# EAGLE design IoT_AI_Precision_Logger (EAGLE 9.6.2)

## Sheet 1 of 4: ADC, Buff Amp, VREF Circuits
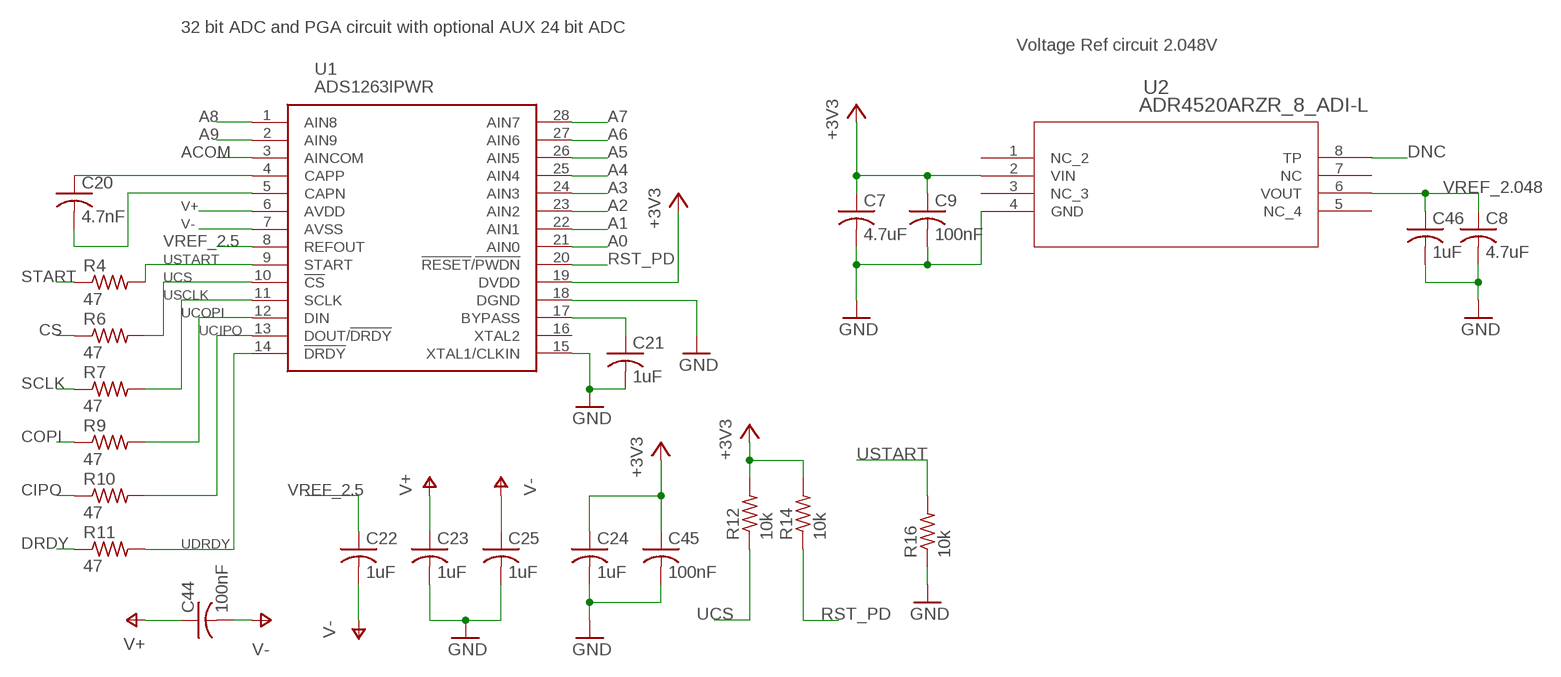
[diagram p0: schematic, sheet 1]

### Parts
C7  4.7uF  C-USC0603  [C0603]
C8  4.7uF  C-USC0603  [C0603]
C9  100nF  C-USC0603  [C0603]
C20  4.7nF  C-USC0603  [C0603]
C21  1uF  C-USC0603  [C0603]
C22  1uF  C-USC0603  [C0603]
C23  1uF  C-USC0603  [C0603]
C24  1uF  C-USC0603  [C0603]
C25  1uF  C-USC0603  [C0603]
C44  100nF  C-USC0603  [C0603]
C45  100nF  C-USC0603  [C0603]
C46  1uF  C-USC0603  [C0603]
R4  47  R-US_R0603  [R0603]
R6  47  R-US_R0603  [R0603]
R7  47  R-US_R0603  [R0603]
R9  47  R-US_R0603  [R0603]
R10  47  R-US_R0603  [R0603]
R11  47  R-US_R0603  [R0603]
R12  10k  R-US_R0603  [R0603]
R14  10k  R-US_R0603  [R0603]
R16  10k  R-US_R0603  [R0603]
U1  ADS1263IPWR  [SOP65P640X120-28N]
U2  ADR4520ARZR_8_ADI-L  [R_8_ADI-L]

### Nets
+3V3: C7.1 C9.1 C24.1 C45.1 R12.2 R14.2 U1.19(DVDD) U2.2(VIN) ; also sheet 2,3,4
A0: U1.21(AIN0) ; also sheet 3
A1: U1.22(AIN1) ; also sheet 3
A2: U1.23(AIN2) ; also sheet 3
A3: U1.24(AIN3) ; also sheet 3
A4: U1.25(AIN4) ; also sheet 3
A5: U1.26(AIN5) ; also sheet 3
A6: U1.27(AIN6) ; also sheet 3
A7: U1.28(AIN7) ; also sheet 3
A8: U1.1(AIN8) ; also sheet 3
A9: U1.2(AIN9) ; also sheet 3
ACOM: U1.3(AINCOM) ; also sheet 3
CIPO: R10.1 ; also sheet 3,4
COPI: R9.1 ; also sheet 4
CS: R6.1 ; also sheet 4
DNC: U2.8(TP)
DRDY: R11.1 ; also sheet 4
GND: C7.2 C8.2 C9.2 C21.2 C23.2 C24.2 C25.2 C45.2 C46.2 R16.1 U1.15(XTAL1/CLKIN) U1.18(DGND) U2.4(GND) ; also sheet 2,3,4
N$8: C20.1 U1.4(CAPP)
N$9: C20.2 U1.5(CAPN)
N$28: C21.1 U1.17(BYPASS)
RST_PD: R14.1 U1.20(!RESET!/!PWDN) ; also sheet 4
SCLK: R7.1 ; also sheet 4
START: R4.1 ; also sheet 4
UCIPO: R10.2 U1.13(DOUT/!DRDY)
UCOPI: R9.2 U1.12(DIN) ; also sheet 3
UCS: R6.2 R12.1 U1.10(!CS)
UDRDY: R11.2 U1.14(!DRDY)
USCLK: R7.2 U1.11(SCLK) ; also sheet 3
USTART: R4.2 R16.2 U1.9(START)
V+: C23.1 C44.1 U1.6(AVDD) ; also sheet 2
V-: C22.2 C25.1 C44.2 U1.7(AVSS) ; also sheet 2,3
VREF_2.5: C22.1 U1.8(REFOUT) ; also sheet 3
VREF_2.048: C8.1 C46.1 U2.6(VOUT) ; also sheet 3
Unconnected: U1.16(XTAL2) U2.1(NC_2) U2.3(NC_3) U2.5(NC_4) U2.7(NC)

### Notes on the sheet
- 32 bit ADC and PGA circuit with optional AUX 24 bit ADC
- Voltage Ref circuit 2.048V

## Sheet 2 of 4: Onboard Power Circuits
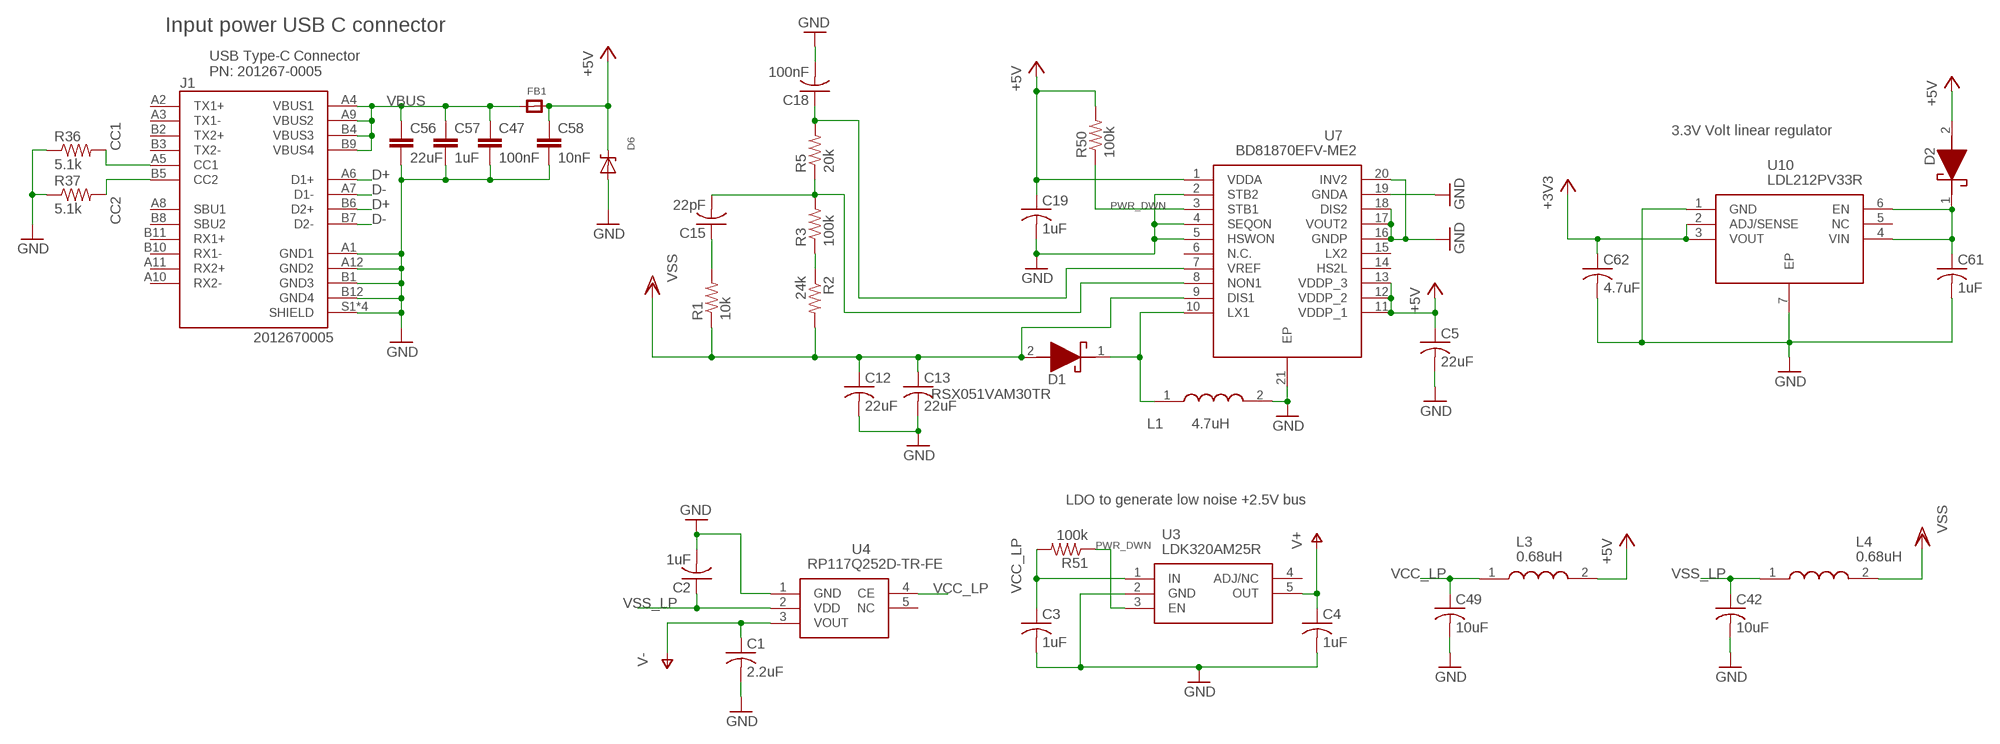
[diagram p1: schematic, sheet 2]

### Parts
C1  2.2uF  C-USC0603  [C0603]
C2  1uF  C-USC0603  [C0603]
C3  1uF  C-USC0603  [C0603]
C4  1uF  C-USC0603  [C0603]
C5  22uF  C-USC0603  [C0603]
C12  22uF  C-USC0603  [C0603]
C13  22uF  C-USC0603  [C0603]
C15  22pF  C-USC0603  [C0603]
C18  100nF  C-USC0603  [C0603]
C19  1uF  C-USC0603  [C0603]
C42  10uF  C-USC0603  [C0603]
C47  100nF  C-EUC0603  [C0603]
C49  10uF  C-USC0603  [C0603]
C56  22uF  C-EUC0603  [C0603]
C57  1uF  C-EUC0603  [C0603]
C58  10nF  C-EUC0603  [C0603]
C61  1uF  C-USC0603  [C0603]
C62  4.7uF  C-USC0603  [C0603]
D1  RSX051VAM30TR  [RSX051VAM30TR]
D2  CUS10S30,H3F  [CUZ10V]
D6  DDZ5V6ASF  [DDZ5V6ASF]
FB1  FERRITE_0603  [_0603]
J1  2012670005  [MOLEX_2012670005]
L1  4.7uH  LQM21PN4R7MGSD  [LQM21PHR47NG0D]
L3  0.68uH  MLF2012DR68MT000  [INDC2012X145N]
L4  0.68uH  MLF2012DR68MT000  [INDC2012X145N]
R1  10k  R-US_R0603  [R0603]
R2  24k  R-US_R0603  [R0603]
R3  100k  R-US_R0603  [R0603]
R5  20k  R-US_R0603  [R0603]
R36  5.1k  R-US_R0603  [R0603]
R37  5.1k  R-US_R0603  [R0603]
R50  100k  R-US_R0603  [R0603]
R51  100k  R-US_R0603  [R0603]
U3  LDK320AM25R  [SOT95P280X125-5N]
U4  RP117Q252D-TR-FE  [SOT65P210X110-5N]
U7  BD81870EFV-ME2  [SOP65P640X100-21N]
U10  LDL212PV33R  [SON50P200X200X80-7N]

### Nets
+3V3: C62.1 U10.2(ADJ/SENSE) U10.3(VOUT) ; also sheet 1,3,4
+5V: C5.1 C19.1 C58.1 D2.2(A) D6.P$2(C) FB1.2 L3.2 R50.2 U7.1(VDDA) U7.11(VDDP_1) U7.12(VDDP_2) U7.13(VDDP_3) ; also sheet 4
CC1: J1.A5(CC1) R36.2
CC2: J1.B5(CC2) R37.2
D+: J1.A6(D1+) J1.B6(D2+) ; also sheet 4
D-: J1.A7(D1-) J1.B7(D2-) ; also sheet 4
GND: C1.2 C2.2 C3.2 C4.2 C5.2 C12.2 C13.2 C18.2 C19.2 C42.2 C47.2 C49.2 C56.2 C57.2 C58.2 C61.2 C62.2 D6.P$1(A) J1.A1(GND1) J1.A12(GND2) J1.B1(GND3) J1.B12(GND4) J1.S1(SHIELD) J1.S2(SHIELD) J1.S3(SHIELD) J1.S4(SHIELD) L1.2 R36.1 R37.1 U3.2(GND) U4.1(GND) U7.2(STB2) U7.4(SEQON) U7.5(HSWON) U7.16(GNDP) U7.17(VOUT2) U7.18(DIS2) U7.19(GNDA) U7.20(INV2) U7.21(EP) U10.1(GND) U10.7(EP) ; also sheet 1,3,4
N$1: C61.1 D2.1(K) U10.4(VIN) U10.6(EN)
N$4: C15.2 R3.2 R5.1 U7.8(NON1)
N$5: D1.1(K) L1.1 U7.10(LX1)
N$6: C18.1 R5.2 U7.7(VREF)
N$7: C15.1 R1.2
N$11: R2.1 R3.1
PWR_DWN: R50.1 R51.1 U3.3(EN) U7.3(STB1) ; also sheet 4
V+: C4.1 U3.5(OUT) ; also sheet 1
V-: C1.1 U4.3(VOUT) ; also sheet 1,3
VBUS: C47.1 C56.1 C57.1 FB1.1 J1.A4(VBUS1) J1.A9(VBUS2) J1.B4(VBUS3) J1.B9(VBUS4) ; also sheet 3
VCC_LP: C3.1 C49.1 L3.1 R51.2 U3.1(IN) U4.4(CE)
VSS: C12.1 C13.1 D1.2(A) L4.2 R1.1 R2.2 U7.9(DIS1)
VSS_LP: C2.1 C42.1 L4.1 U4.2(VDD)
Unconnected: J1.A2(TX1+) J1.A3(TX1-) J1.A8(SBU1) J1.A10(RX2-) J1.A11(RX2+) J1.B2(TX2+) J1.B3(TX2-) J1.B8(SBU2) J1.B10(RX1-) J1.B11(RX1+) U3.4(ADJ/NC) U4.5(NC) U7.6(N.C.) U7.14(HS2L) U7.15(LX2) U10.5(NC)

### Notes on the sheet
- Input power USB C connector
- USB Type-C Connector
  PN: 201267-0005
- 3.3V Volt linear regulator
- LDO to generate low noise +2.5V bus

## Sheet 3 of 4: Connectors and Switching
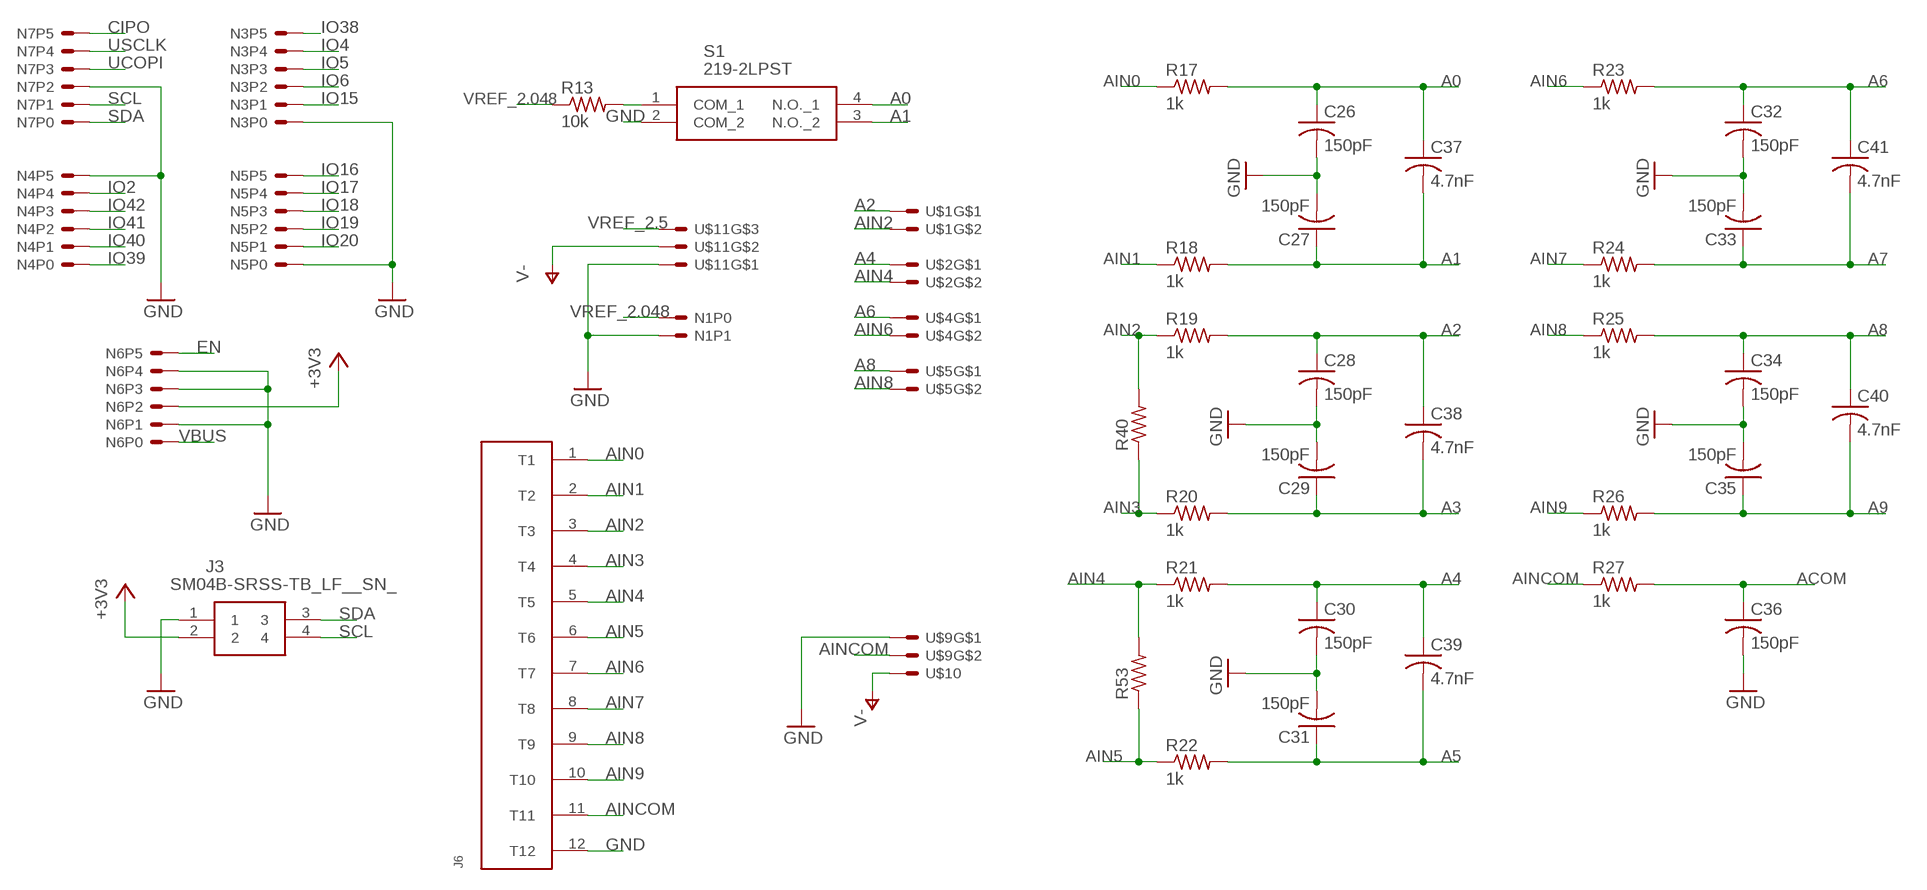
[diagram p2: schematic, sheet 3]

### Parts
C26  150pF  C-USC0603  [C0603]
C27  150pF  C-USC0603  [C0603]
C28  150pF  C-USC0603  [C0603]
C29  150pF  C-USC0603  [C0603]
C30  150pF  C-USC0603  [C0603]
C31  150pF  C-USC0603  [C0603]
C32  150pF  C-USC0603  [C0603]
C33  150pF  C-USC0603  [C0603]
C34  150pF  C-USC0603  [C0603]
C35  150pF  C-USC0603  [C0603]
C36  150pF  C-USC0603  [C0603]
C37  4.7nF  C-USC0603  [C0603]
C38  4.7nF  C-USC0603  [C0603]
C39  4.7nF  C-USC0603  [C0603]
C40  4.7nF  C-USC0603  [C0603]
C41  4.7nF  C-USC0603  [C0603]
J3  SM04B-SRSS-TB_LF__SN_  [SM04B-SRSS-TB(LFSN)]
J6  BARRIER_BLOCK_12POS  [BARRIER_BLOCK_12POS]
N1  2PINHEADER  [2PINHEADER]
N3  6PINHEADER  [6PINHEADER]
N4  6PINHEADER  [6PINHEADER]
N5  6PINHEADER  [6PINHEADER]
N6  6PINHEADER  [6PINHEADER]
N7  6PINHEADER  [6PINHEADER]
R13  10k  R-US_R0603  [R0603]
R17  1k  R-US_R0603  [R0603]
R18  1k  R-US_R0603  [R0603]
R19  1k  R-US_R0603  [R0603]
R20  1k  R-US_R0603  [R0603]
R21  1k  R-US_R0603  [R0603]
R22  1k  R-US_R0603  [R0603]
R23  1k  R-US_R0603  [R0603]
R24  1k  R-US_R0603  [R0603]
R25  1k  R-US_R0603  [R0603]
R26  1k  R-US_R0603  [R0603]
R27  1k  R-US_R0603  [R0603]
R40  R-US_R1206  [R1206]
R53  R-US_R1206  [R1206]
S1  219-2LPST  [2192LPST]
U$1  2PINHEADER_S  [2PINHEADER_S]
U$2  2PINHEADER_S  [2PINHEADER_S]
U$4  2PINHEADER_S  [2PINHEADER_S]
U$5  2PINHEADER_S  [2PINHEADER_S]
U$9  2PINHEADER_S  [2PINHEADER_S]
U$10  1PINHEADER_S  [1PINHEADER_S]
U$11  3PINHEADER  [3PINHEADER]

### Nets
+3V3: J3.2 N6.P2 ; also sheet 1,2,4
A0: C26.1 C37.1 R17.2 S1.4(N.O._1) ; also sheet 1
A1: C27.1 C37.2 R18.2 S1.3(N.O._2) ; also sheet 1
A2: C28.1 C38.1 R19.2 U$1.N0 ; also sheet 1
A3: C29.1 C38.2 R20.2 ; also sheet 1
A4: C30.1 C39.1 R21.2 U$2.N0 ; also sheet 1
A5: C31.1 C39.2 R22.2 ; also sheet 1
A6: C32.1 C41.1 R23.2 U$4.N0 ; also sheet 1
A7: C33.1 C41.2 R24.2 ; also sheet 1
A8: C34.1 C40.1 R25.2 U$5.N0 ; also sheet 1
A9: C35.1 C40.2 R26.2 ; also sheet 1
ACOM: C36.1 R27.2 ; also sheet 1
AIN0: J6.1(T1) R17.1
AIN1: J6.2(T2) R18.1
AIN2: J6.3(T3) R19.1 R40.2 U$1.N1
AIN3: J6.4(T4) R20.1 R40.1
AIN4: J6.5(T5) R21.1 R53.2 U$2.N1
AIN5: J6.6(T6) R22.1 R53.1
AIN6: J6.7(T7) R23.1 U$4.N1
AIN7: J6.8(T8) R24.1
AIN8: J6.9(T9) R25.1 U$5.N1
AIN9: J6.10(T10) R26.1
AINCOM: J6.11(T11) R27.1 U$9.N1
CIPO: N7.P5 ; also sheet 1,4
EN: N6.P5 ; also sheet 4
GND: C26.2 C27.2 C28.2 C29.2 C30.2 C31.2 C32.2 C33.2 C34.2 C35.2 C36.2 J3.1 J6.12(T12) N1.P1 N3.P0 N4.P5 N5.P0 N6.P1 N6.P3 N6.P4 N7.P2 S1.2(COM_2) U$9.N0 U$11.N0 ; also sheet 1,2,4
IO2: N4.P4 ; also sheet 4
IO4: N3.P4 ; also sheet 4
IO5: N3.P3 ; also sheet 4
IO6: N3.P2 ; also sheet 4
IO15: N3.P1 ; also sheet 4
IO16: N5.P5 ; also sheet 4
IO17: N5.P4 ; also sheet 4
IO18: N5.P3 ; also sheet 4
IO19: N5.P2 ; also sheet 4
IO20: N5.P1 ; also sheet 4
IO38: N3.P5 ; also sheet 4
IO39: N4.P0 ; also sheet 4
IO40: N4.P1 ; also sheet 4
IO41: N4.P2 ; also sheet 4
IO42: N4.P3 ; also sheet 4
N$2: R13.2 S1.1(COM_1)
SCL: J3.4 N7.P1 ; also sheet 4
SDA: J3.3 N7.P0 ; also sheet 4
UCOPI: N7.P3 ; also sheet 1
USCLK: N7.P4 ; also sheet 1
V-: U$10.P$1(S) U$11.N1 ; also sheet 1,2
VBUS: N6.P0 ; also sheet 2
VREF_2.5: U$11.N2 ; also sheet 1
VREF_2.048: N1.P0 R13.1 ; also sheet 1

## Sheet 4 of 4: ESP32 Circuit
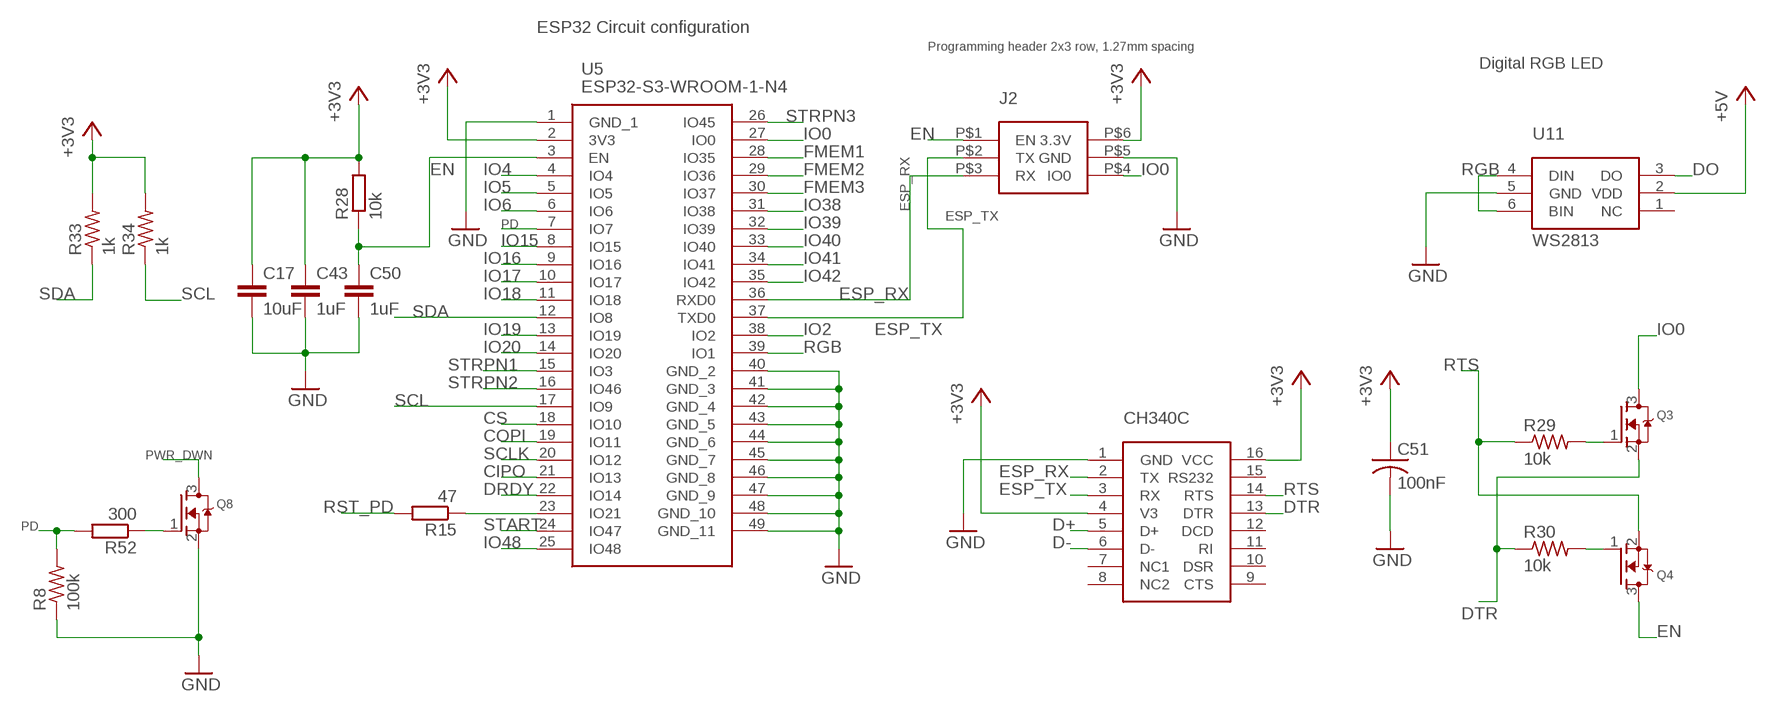
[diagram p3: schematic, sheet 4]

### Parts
C17  10uF  C-EUC0603  [C0603]
C43  1uF  C-EUC0603  [C0603]
C50  1uF  C-EUC0603  [C0603]
C51  100nF  C-USC0603  [C0603]
J2  ESP-PROG_HEADER  [2X3_1.27_HEADER]
Q3  MOSFET-NREFLOW  [SOT23-R]
Q4  MOSFET-NREFLOW  [SOT23-R]
Q8  MOSFET-NREFLOW  [SOT23-R]
R8  100k  R-US_R0603  [R0603]
R15  47  R-EU_R0603  [R0603]
R28  10k  R-EU_R0603  [R0603]
R29  10k  R-US_R0603  [R0603]
R30  10k  R-US_R0603  [R0603]
R33  1k  R-US_R0603  [R0603]
R34  1k  R-US_R0603  [R0603]
R52  300  R-EU_R0603  [R0603]
U5  ESP32-S3-WROOM-1-N4  [ESP32S3WROOM1N4]
U6  CH340C  [SOIC16]
U11  WS2813  [WS2813]

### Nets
+3V3: C17.1 C43.1 C51.1 J2.P$6(3.3V) R28.2 R33.2 R34.2 U5.2(3V3) U6.4(V3) U6.16(VCC) ; also sheet 1,2,3
+5V: U11.2(VDD) ; also sheet 2
CIPO: U5.21(IO13) ; also sheet 1,3
COPI: U5.19(IO11) ; also sheet 1
CS: U5.18(IO10) ; also sheet 1
D+: U6.5(D+) ; also sheet 2
D-: U6.6(D-) ; also sheet 2
DO: U11.3(DO)
DRDY: U5.22(IO14) ; also sheet 1
DTR: Q3.2(S) R30.1 U6.13(DTR)
EN: C50.1 J2.P$1(EN) Q4.3(D) R28.1 U5.3(EN) ; also sheet 3
ESP_RX: J2.P$3(RX) U5.36(RXD0) U6.2(TX)
ESP_TX: J2.P$2(TX) U5.37(TXD0) U6.3(RX)
FMEM1: U5.28(IO35)
FMEM2: U5.29(IO36)
FMEM3: U5.30(IO37)
GND: C17.2 C43.2 C50.2 C51.2 J2.P$5(GND) Q8.2(S) R8.1 U5.1(GND_1) U5.40(GND_2) U5.41(GND_3) U5.42(GND_4) U5.43(GND_5) U5.44(GND_6) U5.45(GND_7) U5.46(GND_8) U5.47(GND_9) U5.48(GND_10) U5.49(GND_11) U6.1(GND) U11.5(GND) ; also sheet 1,2,3
IO0: J2.P$4(IO0) Q3.3(D) U5.27(IO0)
IO2: U5.38(IO2) ; also sheet 3
IO4: U5.4(IO4) ; also sheet 3
IO5: U5.5(IO5) ; also sheet 3
IO6: U5.6(IO6) ; also sheet 3
IO15: U5.8(IO15) ; also sheet 3
IO16: U5.9(IO16) ; also sheet 3
IO17: U5.10(IO17) ; also sheet 3
IO18: U5.11(IO18) ; also sheet 3
IO19: U5.13(IO19) ; also sheet 3
IO20: U5.14(IO20) ; also sheet 3
IO38: U5.31(IO38) ; also sheet 3
IO39: U5.32(IO39) ; also sheet 3
IO40: U5.33(IO40) ; also sheet 3
IO41: U5.34(IO41) ; also sheet 3
IO42: U5.35(IO42) ; also sheet 3
IO48: U5.25(IO48)
N$3: Q4.1(G) R30.2
N$10: Q3.1(G) R29.2
N$17: R15.1 U5.23(IO21)
N$24: Q8.1(G) R52.1
PD: R8.2 R52.2 U5.7(IO7)
PWR_DWN: Q8.3(D) ; also sheet 2
RGB: U5.39(IO1) U11.4(DIN) U11.6(BIN)
RST_PD: R15.2 ; also sheet 1
RTS: Q4.2(S) R29.1 U6.14(RTS)
SCL: R34.1 U5.17(IO9) ; also sheet 3
SCLK: U5.20(IO12) ; also sheet 1
SDA: R33.1 U5.12(IO8) ; also sheet 3
START: U5.24(IO47) ; also sheet 1
STRPN1: U5.15(IO3)
STRPN2: U5.16(IO46)
STRPN3: U5.26(IO45)
Unconnected: U6.7(NC1) U6.8(NC2) U6.9(CTS) U6.10(DSR) U6.11(RI) U6.12(DCD) U6.15(RS232) U11.1(NC)

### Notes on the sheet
- ESP32 Circuit configuration
- Programming header 2x3 row, 1.27mm spacing
- Digital RGB LED
- CH340C

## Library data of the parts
C1-C5 C7-C9 C12 C13 C15 C18-C42 C44-C46 C49 C51 C61 C62 = rcl:C-US: CAPACITOR, American symbol; SPICEPREFIX: C
C17 C43 C47 C50 C56-C58 = rcl:C-EU: CAPACITOR, European symbol; SPICEPREFIX: C
D1 = SamacSys_Parts:RSX051VAM30TR: ROHM 30V 500mA, SiC Schottky Diode, 2-Pin SOD-323HE RSX051VAM30TR; DESCRIPTION: ROHM 30V 500mA, SiC Schottky Diode, 2-Pin SOD-323HE RSX051VAM30TR; HEIGHT: 0.8mm; MANUFACTURER_NAME: ROHM Semiconductor; MANUFACTURER_PART_NUMBER: RSX051VAM30TR; MOUSER_PART_NUMBER: 755-RSX051VAM30TR; MOUSER_PRICE-STOCK: https://www.mouser.co.uk/ProductDetail/ROHM-Semiconductor/RSX051VAM30TR?qs=4v%252BiZTmLVHH6gyykIHF0SA%3D%3D
D2 = SamacSys_Parts:CUS10S30,H3F: Schottky Diodes & Rectifiers Single High-speed switching; DESCRIPTION: Schottky Diodes & Rectifiers Single High-speed switching; HEIGHT: 1.1mm; MANUFACTURER_NAME: Toshiba; MANUFACTURER_PART_NUMBER: CUS10S30,H3F; MOUSER_PART_NUMBER: 757-CUS10S30H3F; MOUSER_PRICE-STOCK: https://www.mouser.co.uk/ProductDetail/Toshiba/CUS10S30H3F?qs=cW4DzVrAanO4Xm6ySrHr7g%3D%3D
D6 = ForceTronics:DDZ5V6ASF: DDZ5V6ASF 5.42 Zener Diode
FB1 = microbuilder:FERRITE: Ferrite Bead
J1 = 2012670005:2012670005: USB-C (USB TYPE-C) USB 3.1 (USB 3.1 Gen 2, Superspeed+) Receptacle Connector 24 Position Surface Mount, Right Angle; Through Hole Check availability; AVAILABILITY: In Stock; DESCRIPTION: USB-C (USB TYPE-C) USB 3.2 Gen 2 (USB 3.1 Gen 2, Superspeed + (USB 3.1)) Receptacle Connector 24 Position Surface Mount, Right Angle; Through Hole; MF: Molex; MP: 2012670005; PACKAGE: None; PRICE: None; PURCHASE-URL: https://pricing.snapeda.com/search/part/2012670005/?ref=eda
J2 = ForceTronics:ESP-PROG_HEADER: 2x3 programming header for the ESP32 with 1.27mm spacing
J3 = SamacSys_Parts:SM04B-SRSS-TB_LF__SN_: JST (JAPAN SOLDERLESS TERMINALS) - SM04B-SRSS-TB(LF)(SN) - CONNECTOR, HEADER, SMT, R/A, 1MM, 4WAY Source: Datasheet; DESCRIPTION: JST (JAPAN SOLDERLESS TERMINALS) - SM04B-SRSS-TB(LF)(SN) - CONNECTOR, HEADER, SMT, R/A, 1MM, 4WAY; HEIGHT: mm; MANUFACTURER_NAME: JST (JAPAN SOLDERLESS TERMINALS); MANUFACTURER_PART_NUMBER: SM04B-SRSS-TB(LF)(SN); MOUSER_PART_NUMBER: 306-SM04BSRSSTBLFSN; MOUSER_PRICE-STOCK: https://www.mouser.co.uk/ProductDetail/JST-Commercial/SM04B-SRSS-TBLFSN?qs=cdbOS8ANM9B3FdyA6cNU2A%3D%3D
J6 = ForceTronics-ForceTronics:BARRIER_BLOCK_12POS: 1 Row 12 positon 7.62mm pin spacing Barrier Bar from Amazon
L1 = SamacSys_Parts:LQM21PN4R7MGSD: LQM21PN_GS Series Inductor 4.7uH +/-20% 0805 (2012); DESCRIPTION: LQM21PN_GS Series Inductor 4.7uH +/-20% 0805 (2012); HEIGHT: 1mm; MANUFACTURER_NAME: Murata Electronics; MANUFACTURER_PART_NUMBER: LQM21PN4R7MGSD; MOUSER_PART_NUMBER: 81-LQM21PN4R7MGSD; MOUSER_PRICE-STOCK: https://www.mouser.co.uk/ProductDetail/Murata-Electronics/LQM21PN4R7MGSD?qs=Gufeu08L%2Fl2uzbzo%2FrY4bg%3D%3D
L3 L4 = SamacSys_Parts:MLF2012DR68MT000: SMD / SMT Inductors (Coils), L=0.68?H, L x W x T :; DESCRIPTION: SMD / SMT Inductors (Coils), L=0.68?H, L x W x T :; HEIGHT: 1.45mm; MANUFACTURER_NAME: TDK; MANUFACTURER_PART_NUMBER: MLF2012DR68MT000
N1 = ForceTronics:2PINHEADER
N3-N7 = ForceTronics:6PINHEADER
Q3 Q4 Q8 = microbuilder:MOSFET-N: N-Channel Mosfet LEGEND VDS: Voltage Drain-Source ID: Drain Current RDS(ON): Drain-Source On-State Resistance VGS(TH): Gate-Source Threshold Voltage CISS: Drain-Source Input Capacitance SOT-23 Name VDS ID RDS(ON) VGS(TH) CISS Order Number 2N7002E 60V 260mA 2.5 Ohm 2.5V @ 250uA 26.7pF @ 25V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
R1-R14 R16-R27 R29 R30 R33 R34 R36 R37 R40 R50 R51 R53 = rcl:R-US_: RESISTOR, American symbol; SPICEPREFIX: R
R15 R28 R52 = rcl:R-EU_: RESISTOR, European symbol; SPICEPREFIX: R
S1 = SamacSys_Parts:219-2LPST: Dip Switch SPST 2 Position Surface Mount Slide (Standard) Actuator 100mA 20VDC Source: Datasheet; DESCRIPTION: Dip Switch SPST 2 Position Surface Mount Slide (Standard) Actuator 100mA 20VDC; HEIGHT: mm; MANUFACTURER_NAME: CTS; MANUFACTURER_PART_NUMBER: 219-2LPST; MOUSER_PART_NUMBER: 774-2192LPST; MOUSER_PRICE-STOCK: https://www.mouser.co.uk/ProductDetail/CTS-Electronic-Components/219-2LPST?qs=qNzHFtQhdJ96rtXqLWSQzw%3D%3D
U1 = SamacSys_Parts:ADS1263IPWR: 32-Bit, 38kSPS, 10-Ch Delta-Sigma ADC w/ PGA, Voltage Reference, and Aux ADC for Factory Automation Source: Datasheet; DESCRIPTION: 32-Bit, 38kSPS, 10-Ch Delta-Sigma ADC w/ PGA, Voltage Reference, and Aux ADC for Factory Automation; HEIGHT: 1.2mm; MANUFACTURER_NAME: Texas Instruments; MANUFACTURER_PART_NUMBER: ADS1263IPWR; MOUSER_PART_NUMBER: 595-ADS1263IPWR; MOUSER_PRICE-STOCK: https://www.mouser.co.uk/ProductDetail/Texas-Instruments/ADS1263IPWR?qs=GURawfaeGuAEKG2KPkczsw%3D%3D
U2 = ForceTronics:ADR4520ARZ; COPYRIGHT: Copyright (C) 2025 Ultra Librarian. All rights reserved.; MANUFACTURER_PART_NUMBER: ADR4520ARZ; MFR_NAME: Analog Devices Inc
U3 = SamacSys_Parts:LDK320AM25R: 200 mA low quiescent current and high PSRR voltage regulator Source: Datasheet; DESCRIPTION: 200 mA low quiescent current and high PSRR voltage regulator; HEIGHT: 1.25mm; MANUFACTURER_NAME: STMicroelectronics; MANUFACTURER_PART_NUMBER: LDK320AM25R; MOUSER_PART_NUMBER: 511-LDK320AM25R; MOUSER_PRICE-STOCK: https://www.mouser.co.uk/ProductDetail/STMicroelectronics/LDK320AM25R?qs=wd5RIQLrsJiQNxEkfV2I5w%3D%3D
U4 = SamacSys_Parts:RP117Q252D-TR-FE: LDO Voltage Regulators 100 mA LDO Regulator Source: Datasheet; DESCRIPTION: LDO Voltage Regulators 100 mA LDO Regulator; HEIGHT: 1.1mm; MANUFACTURER_NAME: Nisshinbo; MANUFACTURER_PART_NUMBER: RP117Q252D-TR-FE; MOUSER_PART_NUMBER: 848-RP117Q252D-TR-FE; MOUSER_PRICE-STOCK: https://www.mouser.co.uk/ProductDetail/Nisshinbo/RP117Q252D-TR-FE?qs=0lQeLiL1qyb%252B39Gkjsmryg%3D%3D
U5 = ESP32-S3-WROOM-1-N4:ESP32-S3-WROOM-1-N4: WiFi Modules - 802.11 [Engineering Samples] SMD Module, ESP32-S3, 4 MB SPI Flash, PCB Antenna Source: Datasheet; DESCRIPTION: WiFi Modules - 802.11 [Engineering Samples] SMD Module, ESP32-S3, 4 MB SPI Flash, PCB Antenna; HEIGHT: 3.25mm; MANUFACTURER_NAME: Espressif Systems; MANUFACTURER_PART_NUMBER: ESP32-S3-WROOM-1-N4; MOUSER_PART_NUMBER: 356-ESP32-S3WROOM1N4; MOUSER_PRICE-STOCK: https://www.mouser.co.uk/ProductDetail/Espressif-Systems/ESP32-S3-WROOM-1-N4?qs=Li%252BoUPsLEnsO%2FkiJOUK0FQ%3D%3D
U6 = ForceTronics:CH340C: CH340C IC that converts USB to UART
U7 = SamacSys_Parts:BD81870EFV-ME2: ROHM - BD81870EFV-ME2 - DC/DC Switching Regulator, Inverting, Step Up, 2 Output, 2.5V to 5.5VIn, 18V out, 2.1MHz, HTSSOP-20 Source: Datasheet; DESCRIPTION: ROHM - BD81870EFV-ME2 - DC/DC Switching Regulator, Inverting, Step Up, 2 Output, 2.5V to 5.5VIn, 18V out, 2.1MHz, HTSSOP-20; HEIGHT: 1mm; MANUFACTURER_NAME: ROHM Semiconductor; MANUFACTURER_PART_NUMBER: BD81870EFV-ME2; MOUSER_PART_NUMBER: 755-BD81870EFV-ME2; MOUSER_PRICE-STOCK: https://www.mouser.co.uk/ProductDetail/ROHM-Semiconductor/BD81870EFV-ME2/?qs=HXFqYaX1Q2wm5IkeUd4YKg%3D%3D
U10 = SamacSys_Parts:LDL212PV33R: LDO Voltage Regulators VFDFPN 6 2x2x0.75 PITCH 0.5 Source: Datasheet; DESCRIPTION: LDO Voltage Regulators VFDFPN 6 2x2x0.75 PITCH 0.5; HEIGHT: 0.8mm; MANUFACTURER_NAME: STMicroelectronics; MANUFACTURER_PART_NUMBER: LDL212PV33R; MOUSER_PART_NUMBER: 511-LDL212PV33R; MOUSER_PRICE-STOCK: https://www.mouser.co.uk/ProductDetail/STMicroelectronics/LDL212PV33R?qs=5aG0NVq1C4xm%252BbuBme%252BLZw%3D%3D
U11 = ForceTronics:WS2813: WS2813 Intelligent control integrated LED light source Device
U$1 U$2 U$4 U$5 U$9 = ForceTronics:2PINHEADER_S: 2 pin header with round copper
U$10 = ForceTronics:1PINHEADER_S: 1 pin header with round pad
U$11 = ForceTronics:3PINHEADER: 3 pin header with oval copper

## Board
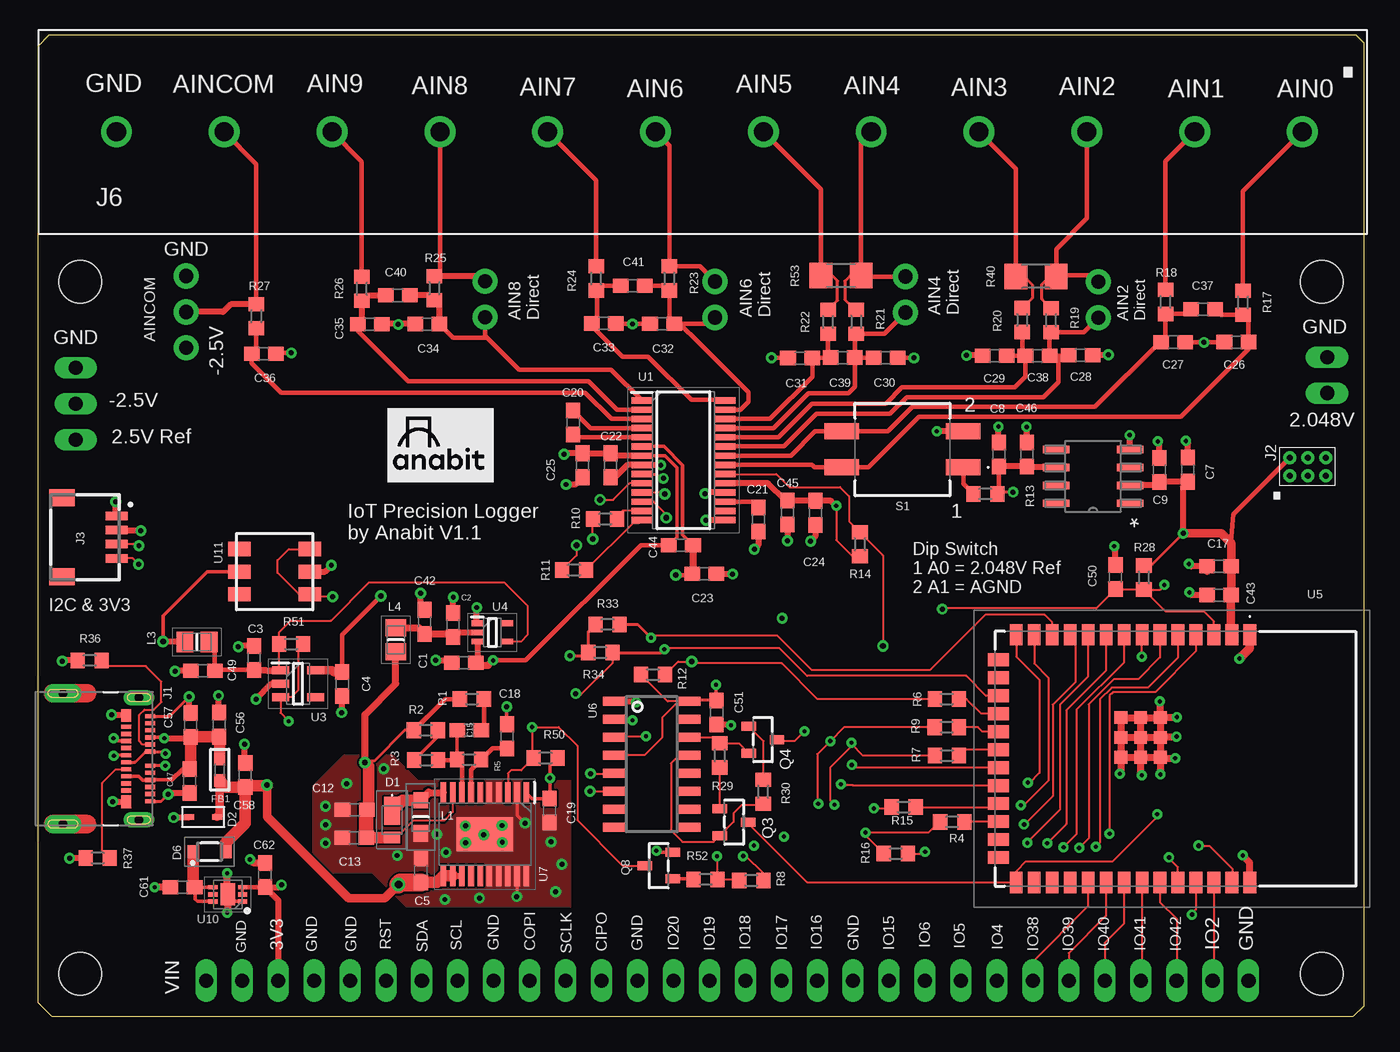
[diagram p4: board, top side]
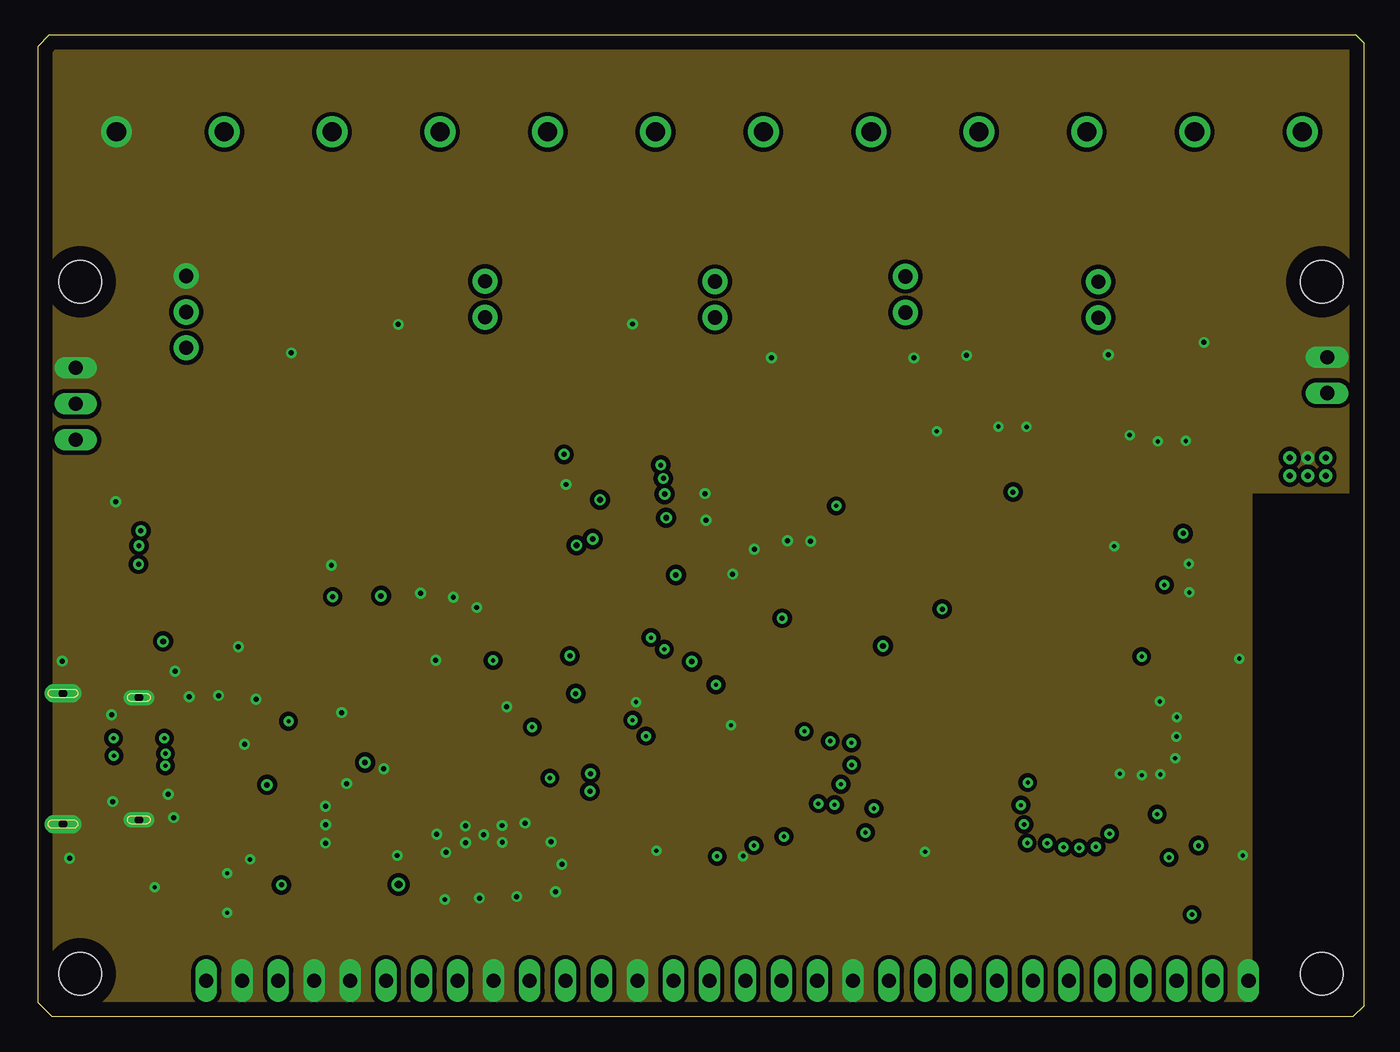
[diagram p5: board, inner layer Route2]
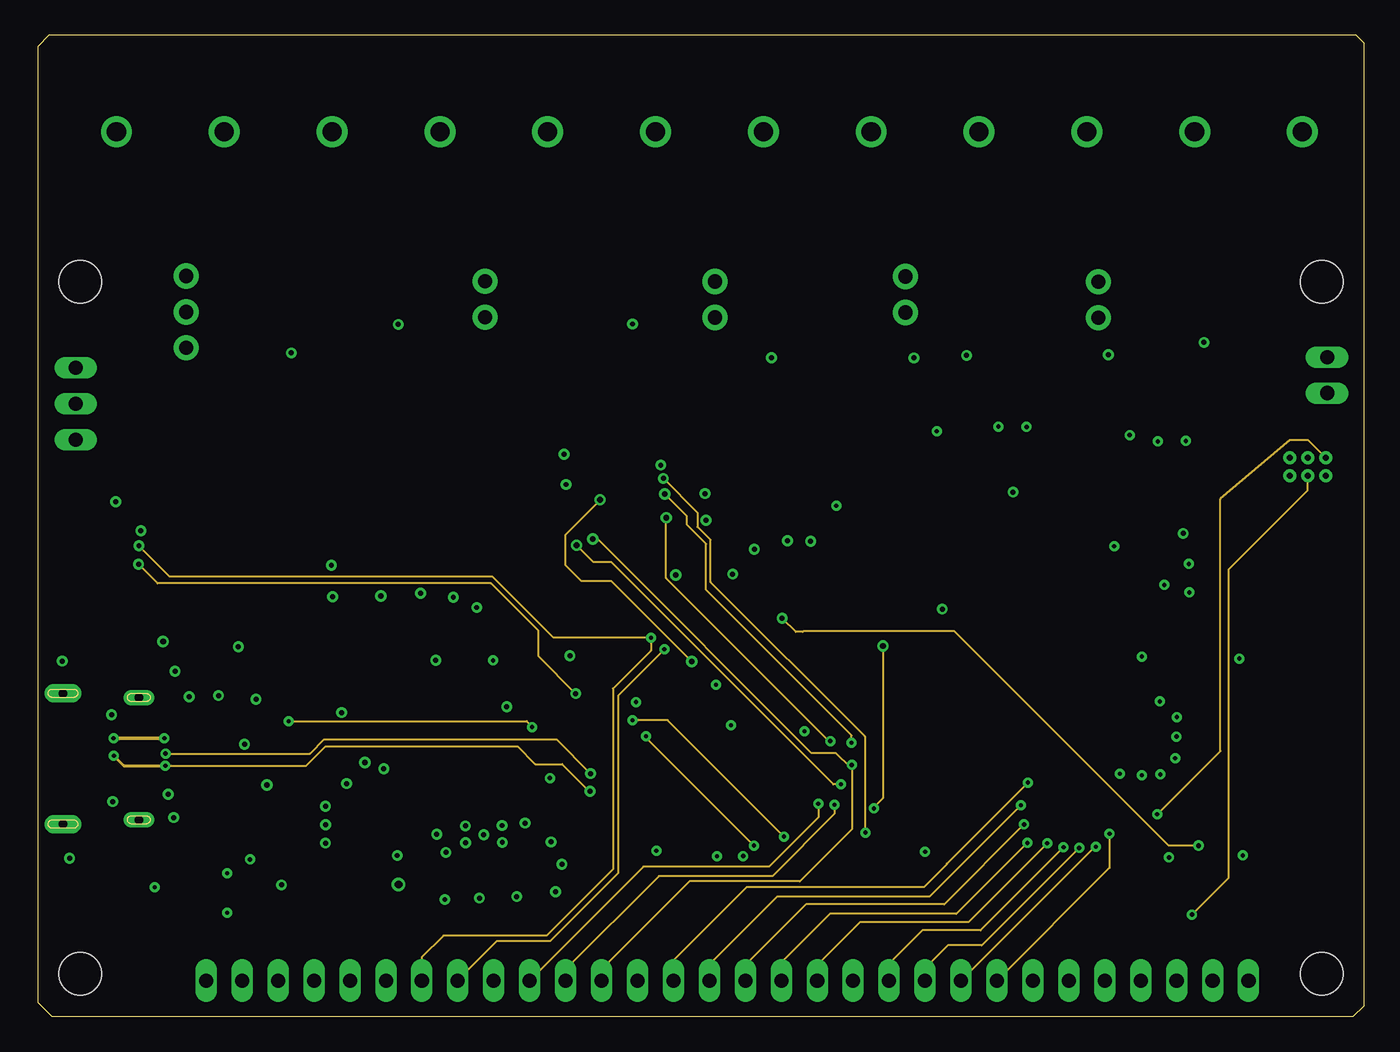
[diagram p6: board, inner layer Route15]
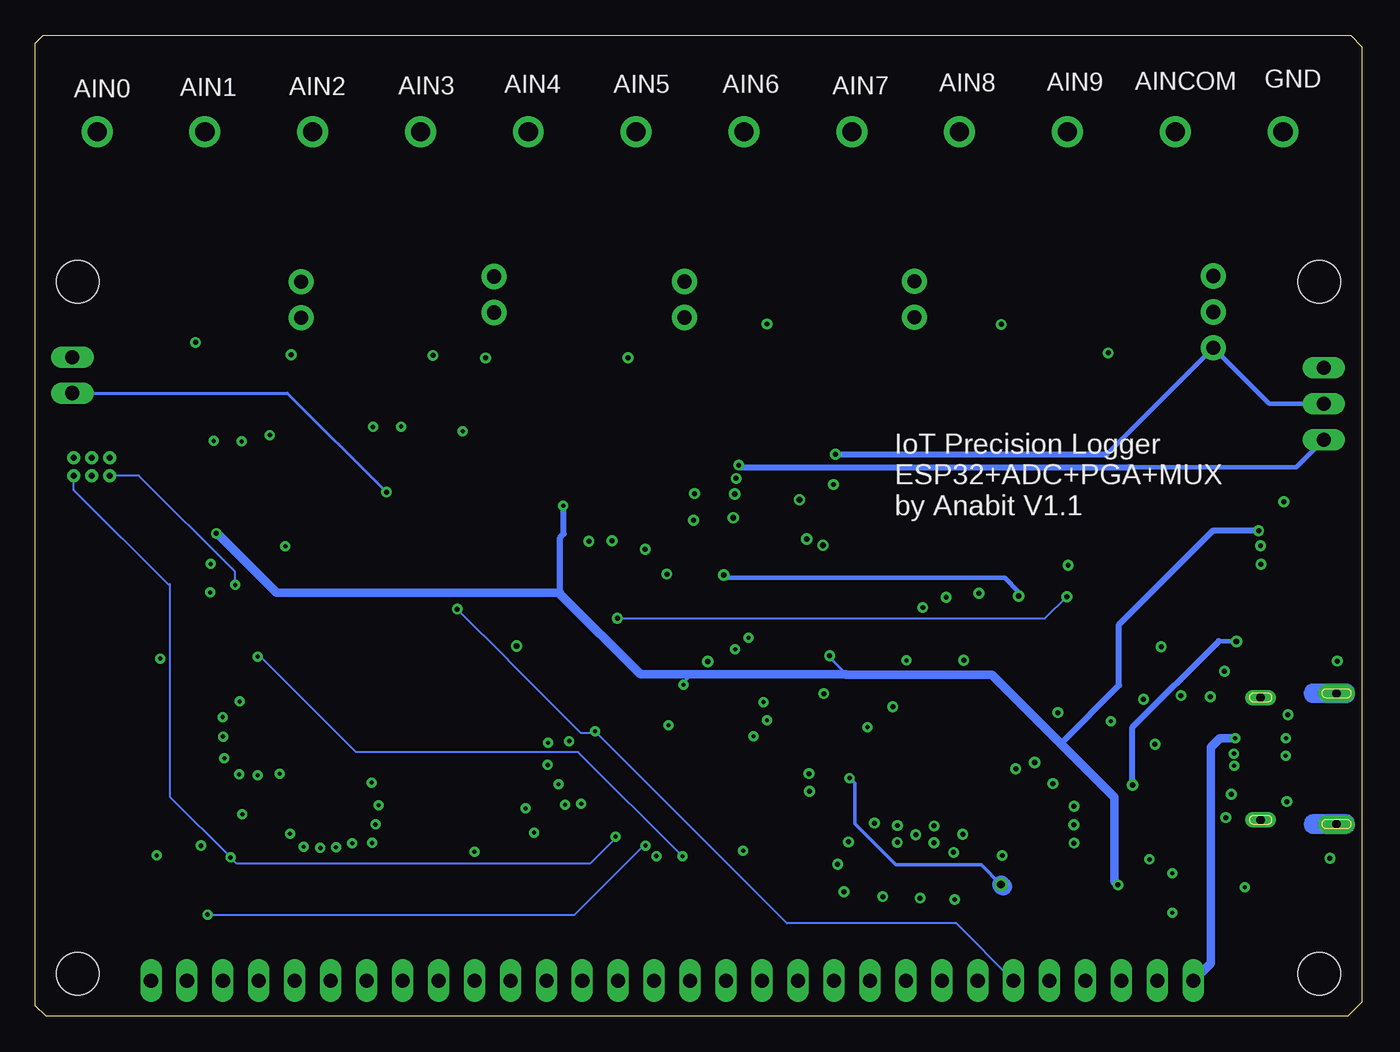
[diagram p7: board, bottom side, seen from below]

Size 93.74 x 69.3 mm. Coordinates in mm from the lower left corner, seen from the top.
Outline: 93.19,69.3 0.79,69.3 0,68.51 0,0.99 0.99,0 92.99,0 93.74,0.75 93.74,68.75 93.19,69.3
Copper layers (1+2*15+16): Top 0.035mm / dielectric 0.5mm / Route2 0.035mm / dielectric 0.75mm / Route15 0.035mm / dielectric 0.75mm / Bottom 0.035mm
Design rules "default *": minimum track width 6mil, minimum drill 0.3mm, track to track 6mil, track to pad 6mil, pad to pad 6mil, via to via 6mil, smd to smd 6mil, copper to edge 40mil, drill to drill 6mil, minimum pad ring 10mil, minimum via ring 8mil, stop-mask expansion 4mil, vias tented up to drill 0mil, thermal gap 10mil
Holes 3 mm at 2.99,51.9 90.75,51.9 2.99,3 90.75,3

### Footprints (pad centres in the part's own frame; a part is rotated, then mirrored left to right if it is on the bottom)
C0603 = smd 1.1 x 1: 1 -0.85,0; 2 0.85,0
RSX051VAM30TR = smd 1.1 x 2: 1 0,0.65 | smd 1.1 x 0.8: 2 0,-1.25
CUZ10V = smd 0.9 x 0.8: 1 0,-1.15; 2 0,1.15
DDZ5V6ASF = smd 0.71 x 0.41: P$1 0,0; P$2 1.99,0
_0603 = smd 0.9 x 0.8: 1 -0.762,0; 2 0.762,0
MOLEX_2012670005 = smd 0.3 x 0.7: A1 -3,0.81; A2 -2.5,0.81; A3 -2,0.81; A4 -1.5,0.81; A5 -1,0.81; A6 -0.5,0.81; A7 0.5,0.81; A8 1,0.81; A9 1.5,0.81; A10 2,0.81; A11 2.5,0.81; A12 3,0.81; B2 2.25,-0.89; B3 1.75,-0.89; B4 1.25,-0.89; B5 0.75,-0.89; B6 0.25,-0.89; B7 -0.25,-0.89; B8 -0.75,-0.89; B9 -1.25,-0.89; B10 -1.75,-0.89; B11 -2.25,-0.89 | smd 0.9 x 0.7: B1 3.05,-0.89; B12 -3.05,-0.89 | drill 0.6 pad 1.1 long: S1 -4.32,0; S2 4.32,0 | drill 0.6 pad 1.3 long: S3 -4.62,-5.36; S4 4.62,-5.36
2X3_1.27_HEADER = drill 0.419 pad 0.75: P$1 0,0; P$2 1.27,0; P$3 2.54,0; P$4 2.54,1.27; P$5 1.27,1.27; P$6 0,1.27
SM04B-SRSS-TB(LFSN) = smd 0.6 x 1.55: 1 1.5,4.661; 2 2.5,4.661; 3 3.5,4.661; 4 4.5,4.661 | smd 1.2 x 1.8: 5 0.2,0.786; 6 5.8,0.786
BARRIER_BLOCK_12POS = drill 1.35 pad 2.184: 1 0,0; 2 7.62,0; 3 15.24,0; 4 22.86,0; 5 30.48,0; 6 38.1,0; 7 45.72,0; 8 53.34,0; 9 60.96,0; 10 68.58,0; 11 76.2,0; 12 83.82,0
LQM21PHR47NG0D = smd 1.15 x 1: 1 -1.175,0; 2 1.175,0
INDC2012X145N = smd 1.2 x 1.45: 1 -0.85,0; 2 0.85,0
2PINHEADER = drill 1 long: P0 -1.27,0; P1 1.27,0
6PINHEADER = drill 1 long: P0 1.27,-1.778; P1 3.81,-1.778; P2 6.35,-1.778; P3 8.89,-1.778; P4 11.43,-1.778; P5 13.97,-1.778
SOT23-R = smd 0.635 x 1.016: 1 -0.95,-1; 2 0.95,-1; 3 0,1
R0603 = smd 1 x 1.1: 1 -0.85,0; 2 0.85,0
R1206 = smd 1.6 x 1.803: 1 -1.422,0; 2 1.422,0
2192LPST = smd 1.13 x 2.44: 1 -1.27,-4.3; 2 1.27,-4.3; 3 1.27,4.3; 4 -1.27,4.3
SOP65P640X120-28N = smd 1.475 x 0.45: 1 -2.938,4.225; 2 -2.938,3.575; 3 -2.938,2.925; 4 -2.938,2.275; 5 -2.938,1.625; 6 -2.938,0.975; 7 -2.938,0.325; 8 -2.938,-0.325; 9 -2.938,-0.975; 10 -2.938,-1.625; 11 -2.938,-2.275; 12 -2.938,-2.925; 13 -2.938,-3.575; 14 -2.938,-4.225; 15 2.938,-4.225; 16 2.938,-3.575; 17 2.938,-2.925; 18 2.938,-2.275; 19 2.938,-1.625; 20 2.938,-0.975; 21 2.938,-0.325; 22 2.938,0.325; 23 2.938,0.975; 24 2.938,1.625; 25 2.938,2.275; 26 2.938,2.925; 27 2.938,3.575; 28 2.938,4.225
R_8_ADI-L = smd 1.876 x 0.508: 1 -2.613,1.905; 2 -2.613,0.635; 3 -2.613,-0.635; 4 -2.613,-1.905; 5 2.613,-1.905; 6 2.613,-0.635; 7 2.613,0.635; 8 2.613,1.905
SOT95P280X125-5N = smd 1.2 x 0.55: 1 -1.25,0.95; 2 -1.25,0; 3 -1.25,-0.95; 4 1.25,-0.95; 5 1.25,0.95
SOT65P210X110-5N = smd 0.85 x 0.4: 1 -1.05,0.65; 2 -1.05,0; 3 -1.05,-0.65; 4 1.05,-0.65; 5 1.05,0.65
ESP32S3WROOM1N4 = smd 1.5 x 0.9: 1 -8.75,5.26; 2 -8.75,3.99; 3 -8.75,2.72; 4 -8.75,1.45; 5 -8.75,0.18; 6 -8.75,-1.09; 7 -8.75,-2.36; 8 -8.75,-3.63; 9 -8.75,-4.9; 10 -8.75,-6.17; 11 -8.75,-7.44; 12 -8.75,-8.71; 13 -8.75,-9.98; 14 -8.75,-11.25; 27 8.75,-11.25; 28 8.75,-9.98; 29 8.75,-8.71; 30 8.75,-7.44; 31 8.75,-6.17; 32 8.75,-4.9; 33 8.75,-3.63; 34 8.75,-2.36; 35 8.75,-1.09; 36 8.75,0.18; 37 8.75,1.45; 38 8.75,2.72; 39 8.75,3.99; 40 8.75,5.26 | smd 0.9 x 1.5: 15 -6.985,-12.5; 16 -5.715,-12.5; 17 -4.445,-12.5; 18 -3.175,-12.5; 19 -1.905,-12.5; 20 -0.635,-12.5; 21 0.635,-12.5; 22 1.905,-12.5; 23 3.175,-12.5; 24 4.445,-12.5; 25 5.715,-12.5; 26 6.985,-12.5 | smd 0.9 x 0.9: 41 -1.5,-2.46; 42 -0.1,-2.46; 43 -0.1,-1.06; 44 -1.5,-1.06; 45 -2.9,-1.06; 46 -2.9,-2.46; 47 -2.9,-3.86; 48 -1.5,-3.86; 49 -0.1,-3.86
SOIC16 = smd 0.635 x 1.524: 1 -4.445,-2.695; 2 -3.175,-2.695; 3 -1.905,-2.695; 4 -0.635,-2.695; 5 0.635,-2.695; 6 1.905,-2.695; 7 3.175,-2.695; 8 4.445,-2.695; 9 4.445,2.695; 10 3.175,2.695; 11 1.905,2.695; 12 0.635,2.695; 13 -0.635,2.695; 14 -1.905,2.695; 15 -3.175,2.695; 16 -4.445,2.695
SOP65P640X100-21N = smd 1.475 x 0.4: 1 -2.938,2.925; 2 -2.938,2.275; 3 -2.938,1.625; 4 -2.938,0.975; 5 -2.938,0.325; 6 -2.938,-0.325; 7 -2.938,-0.975; 8 -2.938,-1.625; 9 -2.938,-2.275; 10 -2.938,-2.925; 11 2.938,-2.925; 12 2.938,-2.275; 13 2.938,-1.625; 14 2.938,-0.975; 15 2.938,-0.325; 16 2.938,0.325; 17 2.938,0.975; 18 2.938,1.625; 19 2.938,2.275; 20 2.938,2.925 | smd 2.4 x 4: 21 0,0
SON50P200X200X80-7N = smd 0.65 x 0.3: 1 -1.05,0.5; 2 -1.05,0; 3 -1.05,-0.5; 4 1.05,-0.5; 5 1.05,0; 6 1.05,0.5 | smd 1.02 x 1.55: 7 0,0
WS2813 = smd 1.6 x 1: 1 5.2,1.1; 2 5.2,2.7; 3 5.2,4.3; 4 0.2,4.3; 5 0.2,2.7; 6 0.2,1.1
2PINHEADER_S = drill 1 pad 1.778: N0 2.59,0.056; N1 0.05,0.056
1PINHEADER_S = drill 1 pad 1.778: P$1 1.27,1.27
3PINHEADER = drill 1 long: N0 1.27,1.27; N1 3.81,1.27; N2 6.35,1.27

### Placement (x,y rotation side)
C1  30.12,24.98 180 top
C2  29.35,27.65 90 top
C3  15.29,25.32 90 top
C4  21.52,23.47 270 top
C5  27.08,10.31 90 top
C7  81.28,38.62 90 top
C8  67.92,39.7 90 top
C9  79.27,38.6 90 top
C12  22.39,14.59 180 top
C13  22.37,12.62 180 top
C15  30.49,20.22 180 top
C17  83.49,31.79 180 top
C18  33.16,19.78 90 top
C19  36.17,14.53 270 top
C20  37.84,41.94 270 top
C21  50.93,35.11 270 top
C22  40.49,38.93 90 top
C23  47.11,31.26 0 top
C24  54.96,35.57 270 top
C25  38.5,38.93 270 top
C26  84.71,47.64 180 top
C27  80.25,47.63 0 top
C28  73.69,46.7 0 top
C29  67.62,46.66 180 top
C30  59.92,46.53 0 top
C31  53.87,46.51 180 top
C32  44.12,48.93 180 top
C33  40,48.94 0 top
C34  27.52,48.91 180 top
C35  23.46,48.89 0 top
C36  15.97,46.8 0 top
C37  82.36,49.96 180 top
C38  70.65,46.66 180 top
C39  56.89,46.54 180 top
C40  25.45,50.93 180 top
C41  42.04,51.61 180 top
C42  27.35,27.87 90 top
C43  83.48,29.76 180 top
C44  45.46,33.29 180 top
C45  52.98,35.59 270 top
C46  69.91,39.7 90 top
C47  10.74,16.62 270 top
C49  11.66,24.41 180 top
C50  76.17,31.03 90 top
C51  47.98,21.47 270 top
C56  12.82,20.6 90 top
C57  10.81,20.57 90 top
C58  14.67,17.04 90 top
C61  10.24,9.11 180 top
C62  16.06,9.97 90 top
D1  25.04,13.87 0 top
D2  12.14,11.63 270 top
D6  10.69,14.08 0 top
FB1  12.86,17.42 270 top
J1  7.14,18.2 270 top
J2  88.48,38.19 0 top
J3  0.91,36.85 270 top
J6  89.38,62.48 180 top
L1  27.07,14.08 270 top
L3  11.25,26.44 180 top
L4  25.3,26.6 270 top
N1  91.13,45.3 90 top
N3  56.35,4.3 0 top
N4  71.6,4.3 0 top
N5  41.12,4.3 0 top
N6  10.64,4.3 0 top
N7  25.87,4.3 0 top
Q3  49.21,13.72 270 top
Q4  51.24,19.54 270 top
Q8  43.89,10.65 90 top
R1  30.68,22.41 0 top
R2  27.43,20.21 180 top
R3  27.44,18.1 0 top
R4  64.63,13.73 180 top
R5  30.49,18.13 0 top
R6  64.25,22.41 180 top
R7  64.25,18.42 180 top
R8  50.43,9.59 180 top
R9  64.24,20.42 180 top
R10  40.1,35.13 0 top
R11  37.9,31.53 0 top
R12  43.48,24.14 180 top
R13  66.97,36.91 180 top
R14  58.11,33.34 270 top
R15  61.2,14.78 180 top
R16  60.64,11.49 180 top
R17  85.18,50.42 270 top
R18  79.7,50.47 270 top
R19  71.61,49.17 270 top
R20  69.58,49.19 270 top
R21  57.85,49.07 270 top
R22  55.85,49.06 270 top
R23  44.64,52.13 270 top
R24  39.46,52.13 270 top
R25  28.04,51.44 270 top
R26  22.9,51.4 270 top
R27  15.45,49.45 270 top
R28  78.17,31 90 top
R29  48.2,18.43 270 top
R30  51.26,15.87 90 top
R33  40.26,27.69 180 top
R34  39.76,25.7 180 top
R36  3.67,25.14 0 top
R37  4.24,11.18 0 top
R40  70.55,52.27 0 top
R50  35.88,18.25 0 top
R51  17.91,26.29 180 top
R52  47.2,9.67 0 top
R53  56.77,52.33 0 top
S1  61.11,40.05 90 top
U1  45.63,39.28 0 top
U2  74.58,38.14 180 top
U3  18.4,23.49 0 top
U4  32.12,27.12 0 top
U5  80.4,18.2 270 top
U6  43.39,17.81 270 top
U7  31.6,12.86 270 top
U10  13.43,8.61 180 top
U11  19.44,34.11 180 top
U$1  74.9,51.94 270 top
U$2  61.27,52.31 270 top
U$4  47.81,51.96 270 top
U$5  31.56,51.97 270 top
U$9  10.55,49.71 90 top
U$10  9.23,45.96 0 top
U$11  1.41,47.08 270 top

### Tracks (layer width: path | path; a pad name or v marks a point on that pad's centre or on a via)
+3V3  (via drill 0.3, 0.35)
  Top 0.152: U6.4 42.88,18.45 44.12,19.69 44.12,21.09 45.29,22.25 U6.16 44.52,22.25 R12.2 | C17.1 84.34,31.74 84.34,31.6 | R14.2 57.57,32.49 56.43,33.63 v56.43,36.06
  Top 0.2: v80.95,34.11 78.69,31.85 R28.2
  Top 0.203: U10.2 U10.3 | C51.1 47.91,22.32 46.15,22.32 U6.16 | v37.61,25.46 38.68,25.46 R34.2 38.91,27.19 R33.2
  Top 0.254: v47.93,23.42 47.93,22.34 47.91,22.32
  Top 0.305: C62.1 U10.3 | C17.1 84.34,33.89 84.51,35.49 J2.P$6
  Top 0.406: v56.43,36.06 56.07,36.42 C24.1 53,36.42 C45.1 52.83,36.44 51.62,37.66 U1.19 | U2.2 79.02,37.51 C9.1 79.27,37.77 C7.1 80.95,37.43 v80.95,34.11 | N6.P2 16.99,8.19 C62.1 17.06,9.12 v17.22,9.28 | v7.29,34.3 5.62,34.3 J3.2
  Top 0.508: C62.1 16.11,9.17
  Top 0.61: v80.95,34.11 83.65,34.11 84.34,33.42 84.34,31.74 | C17.1 C43.1 84.33,27.01 U5.2
  Bottom 0.203: 36.46,24.13 36.46,24.15 36.46,24.21 37.66,25.41 v37.61,25.46
  Bottom 0.254: 47.38,24.15 47.9,23.63 47.9,23.42 v47.93,23.42
  Bottom 0.406: v56.43,36.06 56.4,36.03 56.4,34.08 56.65,33.83 56.65,29.91 56.65,29.79 | 80.9,34.11 v80.95,34.11 | 21.27,19.25 17.16,23.37 17.16,27.67 10.5,34.33 7.29,34.33 v7.29,34.3
  Bottom 0.61: v17.22,9.28 17.49,9.55 17.49,15.47 21.27,19.25 26.15,24.13 36.46,24.13 | 56.65,29.79 56.62,29.79 50.98,24.15 47.38,24.15 36.46,24.15 | 56.65,29.91 76.7,29.91 80.9,34.11
+5V  (via drill 0.3, 0.4, 0.55)
  Top 0.254: U7.1 34.94,15.38 C19.1 36.19,15.4 v36.19,16.83 36.19,17.71 R50.2 | v8.86,26.48 8.86,28.31 11.96,31.41 U11.2
  Top 0.305: 10.36,26.48 L3.2
  Top 0.406: U7.12 U7.13 | v8.86,26.48 10.36,26.48
  Top 0.61: FB1.2 12.86,14.26 D6.P$2 | v16.2,16.35 16.2,14.11 21.97,8.34 24.53,8.34 25.63,9.44
  Top 0.813: C5.1 28.21,9.46 U7.11 U7.12 | FB1.2 13.33,16.19 C58.1 | C58.1 14.67,13.63 13.29,12.25 D2.2 | C58.1 14.76,16.28 16.2,16.28 v16.2,16.35
  Top 1.27: v25.5,9.31 25.63,9.44 27.06,9.44 C5.1
  Bottom 0.254: v25.5,9.31 26.88,10.69 32.93,10.69 35.83,13.59 35.83,16.47 v36.19,16.83
  Bottom 0.305: 10.11,26.51 8.86,26.51 v8.86,26.48
  Bottom 0.406: v16.2,16.35 16.2,20.42 10.11,26.51
  Bottom 1.27: v25.5,9.31 25.35,9.16
A0
  Top 0.305: C37.1 83.6,49.57 R17.2 85.56,49.19 C26.1 85.56,47.12 80.78,42.34 62.26,42.34 58.7,38.78 S1.4 54.9,38.78 54.73,38.95 U1.21
A1
  Top 0.305: C37.2 81.17,49.62 R18.2 79.7,47.93 C27.1 79.29,47.63 74.71,43.05 61.82,43.05 60.09,41.32 S1.3 54.94,41.32 53.23,39.6 U1.22
A2
  Top 0.305: U$1.N0 73.93,48.32 R19.2 71.5,48.21 C38.1 72.14,46.66 | C28.1 72.8,46.66 72.14,46.66 | U1.23 52.73,40.26 55.04,42.56 60.24,42.56 61.42,43.74 71.08,43.74 72.14,44.8 72.14,46.66
A3
  Top 0.305: C38.2 69.58,46.88 R20.2 | C38.2 C29.1 | C38.2 69.8,45.17 69.06,44.43 61.08,44.43 59.93,43.28 54.73,43.28 52.36,40.91 U1.24
A4
  Top 0.305: C39.1 57.74,48.11 R21.2 59.83,48.22 U$2.N0 | C39.1 C30.1 | U1.25 52.01,41.55 54.47,44.02 57.3,44.02 57.76,44.48 57.76,46.52 C39.1
A5
  Top 0.254: 55.97,48.09 R22.2 55.93,48.13 | 55.59,46.54 55.89,46.54 C39.2
  Top 0.305: C31.1 54.75,46.54 | 54.75,46.54 55.89,46.54 | C39.2 55.85,46.73 R22.2 | U1.26 51.76,42.2 54.75,45.2 54.75,46.54
A6
  Top 0.305: C32.1 44.64,49.26 44.64,51.18 | 44.64,51.18 R23.2 | C41.1 44.21,51.61 44.64,51.18 | C32.1 45.37,48.93 46.72,47.58 46.73,47.58 50.24,44.07 50.24,43.43 49.66,42.85 U1.27 | C32.1 47.43,48.93 U$4.N0
A7
  Top 0.254: 41.19,51.96 C41.2 | 39.54,51.05 R24.2
  Top 0.305: C41.2 39.79,51.61 R24.2 39.52,51.22 39.52,49.31 C33.1 | U1.28 48.53,43.55 46.2,43.55 43.13,46.61 41.32,46.61 39.15,48.78 C33.1 | 39.13,48.92 C33.1
A8
  Top 0.254: R25.2 28.09,50.54
  Top 0.305: R25.2 28.37,50.26 | C34.1 29.34,47.94 31.76,47.94 | U1.1 40.51,45.69 34.01,45.69 31.76,47.94 | 31.76,47.94 31.62,48.08 U$5.N0
  Top 0.406: R25.2 27.7,50.93 C40.1 | 28.37,50.26 C34.1
A9
  Top 0.254: 24.6,50.98 C40.2 24.95,50.58 | R26.2 22.83,50.48
  Top 0.305: 22.9,49.18 C35.1 22.61,48.43 26.18,44.86 38.92,44.86 40.93,42.85 U1.2
  Top 0.406: C40.2 23.28,50.93 R26.2 22.9,49.18
ACOM
  Top 0.305: U1.3 40.54,42.2 38.69,44.05 17.19,44.05 15.12,46.12 C36.1 15.45,47.13 R27.2
AIN0
  Top 0.305: J6.1 85.18,58.28 R17.1
AIN1
  Top 0.305: J6.2 79.7,60.42 R18.1
AIN2
  Top 0.2: R19.1 70.97,50.66 70.97,51.71 71.76,52.5 72.38,52.5
  Top 0.305: J6.3 74.14,56.37 71.97,54.2 R40.2 | U$1.N1 74.51,52.34 72.04,52.34 R40.2 | 72.38,52.5 72.15,52.27 R40.2
AIN3
  Top 0.2: R40.1 69.21,52.35 69.62,52.35 70.28,51.69 70.28,50.74 R20.1
  Top 0.305: J6.4 69.13,59.87 R40.1 69.66,51.74
AIN4
  Top 0.2: R53.2 57.43,52.33 57.04,51.94 57.04,50.64 57.76,49.92 R21.1
  Top 0.305: U$2.N1 58.26,52.26 R53.2 58.19,61.77 J6.5
AIN5
  Top 0.2: R22.1 56.52,50.58 56.52,51.95 56.16,52.31 55.37,52.31 R53.1
  Top 0.305: J6.6 55.35,58.41 R53.1
AIN6
  Top 0.305: U$4.N1 46.8,52.98 R23.1 44.64,61.5 J6.7
AIN7
  Top 0.254: R24.1 39.86,53.23
  Top 0.305: R24.1 39.46,59.06 J6.8
AIN8
  Top 0.305: J6.9 28.42,52.67 R25.1
  Top 0.406: U$5.N1 31.25,52.29 R25.1
AIN9
  Top 0.254: R26.1 23.15,52.5
  Top 0.305: J6.10 22.9,60.38 R26.1
AINCOM
  Top 0.305: J6.11 15.45,60.21 R27.1
  Top 0.406: R27.1 13.64,50.3 13.1,49.76 U$9.N1
CC1
  Top 0.152: J1.A5 7.43,19.2 7.17,19.46 7.17,21.3 7.54,21.67 8.21,21.67 8.73,22.19 8.73,23.64 7.63,24.74 4.92,24.74 R36.2
CC2
  Top 0.152: R37.2 4.56,11.71 4.56,16.49 5.52,17.45 J1.B5
CIPO  (via drill 0.3, 0.4)
  Top 0.152: U5.21 57.53,17.57 v57.53,17.76 | v39.22,33.72 39.22,35.1 R10.1
  Route15 0.152: v39.22,33.72 39.32,33.62 39.67,33.62 54.69,18.6 56.41,18.6 57.39,17.62 v57.53,17.76 57.53,13.21 53.85,9.53 46.05,9.53 39.84,3.32 N7.P5
COPI
  Top 0.152: U5.19 66.77,20.11 66.45,20.42 R9.1
CS
  Top 0.152: U5.18 66.67,21.38 65.64,22.41 R6.1
D+  (via drill 0.3, 0.35)
  Top 0.152: v39.07,17.15 40.67,17.15 U6.5
  Top 0.2: J1.B6 6.87,17.95 7.62,18.7 J1.A6 9.01,18.7 9.09,18.62 v9.03,18.56
  Route15 0.152: v9.03,18.56 19.24,18.56 20.24,19.56 36.66,19.56 v39.07,17.15
D-  (via drill 0.3, 0.35)
  Top 0.152: v39.02,15.89 39.04,15.9 U6.6
  Top 0.2: J1.B7 5.42,18.45 v5.38,18.41 | v9.02,17.7 J1.A7
  Route15 0.152: v9.02,17.7 18.98,17.7 20.35,19.07 33.91,19.07 35.16,17.82 37.07,17.82 v39.01,15.88 v39.02,15.89
  Route15 0.2: v5.38,18.41 6.08,17.71 v9.01,17.71 v9.02,17.7
DRDY  (via drill 0.3, 0.4)
  Top 0.152: U5.22 57.64,16.3 57.61,16.32 56.83,16.32 v56.76,16.39 | v38.08,33.28 38.08,32.56 R11.1
  Route15 0.152: v56.76,16.39 56.23,16.39 40.54,32.08 39.28,32.08 v38.08,33.28
DTR
  Top 0.152: U6.13 45.33,18.45 44.74,17.86 44.74,13.15 45.56,12.33 47.77,12.33 Q3.2 49.17,13.73 49.17,14.35 49.74,14.92 51.16,14.92 R30.1
EN  (via drill 0.3, 0.35)
  Top 0.152: 52.24,19.45 Q4.3 52.33,19.45 53.5,19.45 v54.18,20.13 | U5.3 83.12,27.9 82.43,28.59 79.73,28.59 R28.1 | R28.1 76.16,30.15 76.15,30.16 C50.1 74.81,28.82 63.97,28.82 v63.92,28.77 | R28.1 79.35,30.15 79.65,30.45 v79.62,30.48
  Bottom 0.152: v63.92,28.77 60.33,25.18 60.33,25.16 55.2,20.03 54.2,20.03 54.18,20.05 v54.18,20.13 40.62,6.57 28.66,6.57 N6.P5 | v79.62,30.48 79.62,31.39 86.42,38.19 J2.P$1
ESP_RX  (via drill 0.3)
  Top 0.152: v42.04,20.92 v42.03,20.93 40.68,20.93 40.7,20.95 U6.2 | U5.36 80.58,10.53 79.95,11.16 v79.95,11.22
  Route15 0.152: v52.74,12.7 44.52,20.92 v42.04,20.92
  Bottom 0.152: v52.74,12.7 52.68,12.64 54.5,10.82 79.55,10.82 v79.95,11.22 84.22,15.49 84.22,30.37 | 84.22,30.37 84.22,30.53 | 84.22,30.37 91.02,37.17 J2.P$3
ESP_TX  (via drill 0.3)
  Top 0.152: U6.3 40.77,19.79 v42.99,19.79 | U5.37 81.85,7.56 81.53,7.24 v81.58,7.19
  Route15 0.152: v50.62,12.06 42.99,19.69 v42.99,19.79 | v81.58,7.19 84.16,9.77 84.16,31.58 89.75,37.17 J2.P$2
  Bottom 0.152: v81.58,7.19 55.62,7.19 50.75,12.06 v50.62,12.06
GND  (via drill 0.3, 0.35)
  Top 0.152: C34.2 26.61,48.85 25.53,48.85 | R16.1 62.57,11.49 v62.71,11.63 | R8.1 51.28,10.09 50.02,11.35 49.88,11.35 v49.85,11.32
  Top 0.2: J1.A1 9.32,21.2 v10.7,22.58 | J1.A12 8.73,15.2 v9.22,15.69 | v5.29,15.17 5.31,15.15
  Top 0.254: U7.19 33.88,8.46 v33.85,8.46 | U10.1 13.42,8.11 | U7.2 33.88,14.21 v34.44,13.65 | C18.2 33.14,20.65 v33.14,21.87 | Q8.2 43.82,11.6 v43.72,11.7
  Top 0.305: C27.2 82.4,47.63 v82.42,47.61 83.72,47.61 83.77,47.55 C26.2 | C30.2 61.9,46.53 v61.92,46.51 | C31.2 v51.87,46.51 v51.86,46.52 | C32.2 43.25,48.91 v42.04,48.91 42.01,48.94 C33.2 | 24.33,48.91 C35.2 | 25.53,48.85 25.5,48.88 v25.48,48.88 | C36.2 16.89,46.87 v17.92,46.87
  Top 0.406: U3.2 16.51,23.49 v15.42,22.4 | v14.17,26.1 14.06,26.1 13.99,26.17 C3.2 | C4.2 21.45,21.5 v21.48,21.46 | v28.12,25.16 29.1,25.16 C1.2 | C42.2 27.06,29.01 v27.06,29.88 | C2.2 29.35,29.59 v29.37,29.61 | C21.2 50.93,33.29 v50.64,33 | C45.2 v52.98,33.59 | C24.2 54.96,33.9 v54.62,33.56 | U1.15 47.25,35.05 v47.23,35.04 | U1.18 47.23,37.01 v47.16,36.93 | C29.2 66.77,46.69 v65.64,46.69 | C28.2 74.57,46.73 v75.66,46.73 | C34.2 24.33,48.91 | C25.2 37.99,37.57 v37.33,37.57 | U6.1 42.23,22.25 v42.28,22.2 | C51.2 48.94,20.62 v49,20.56 | C23.2 49.09,31.26 v49.11,31.24 | S1.2 63.55,41.32 v63.53,41.34 | C8.2 67.89,40.58 v67.89,41.66 | C46.2 69.91,41.6 v69.88,41.64 | U2.4 77.19,41.04 v77.17,41.06 | C9.2 79.27,40.51 v79.16,40.61 | C7.2 81.28,40.51 v81.14,40.65 | J3.1 5.51,35.41 v5.51,36.35 | R37.1 v2.25,11.17 | R36.1 1.78,25.14 v1.73,25.09 | C43.2 81.56,29.76 v81.38,29.94 | C17.2 81.52,31.79 v81.35,31.96 | C50.2 76.17,33.1 v76.07,33.2 | U11.5 20.3,31.41 v20.75,31.86 | 5.31,15.15 J1.B1 | J1.B12 5.27,21.25 v5.21,21.31 | C49.2 9.73,24.41 v9.7,24.38 | C57.2 10.7,21.53 v10.7,22.58 | C56.2 12.77,21.5 v12.77,22.66 | D6.P$1 10.65,14.04 v9.61,14.04 | C47.2 9.3,15.77 v9.22,15.69 | C58.2 14.61,17.95 v14.61,19.22 | U4.1 31.02,27.82 v31.02,28.88
  Top 0.508: C62.2 15.26,10.82 v15,11.08 | 13.43,8.28 U10.7 13.39,8.65 v13.39,10.11 | 13.42,8.11 13.42,7.35 v13.39,7.32 | C61.2 v8.28,9.11 v8.27,9.12 | C17.2 82.64,31.43 | U5.48 U5.47 U5.46 | U5.48 U5.49 | U5.49 76.54,17.2 v76.48,17.14 | U5.46 U5.41 | U5.41 U5.42 | U5.42 77.94,17.11 v78.03,17.02 | U5.45 U5.44 | U5.44 U5.43 | U5.43 v79.34,17.09 | U5.45 79.34,22.21 v79.31,22.24 | U5.46 U5.45 | U5.45 79.38,21.14 v80.5,21.14 | U5.48 U5.41 | U5.41 U5.44 | U5.44 79.4,19.76 v80.48,19.76 | U5.49 U5.42 | U5.42 U5.43 | U5.43 79.41,18.23 v80.38,18.23 | U5.40 85.66,10.86 v85.16,11.36
  Top 0.61: U5.1 85.66,26.01 v84.92,25.27
  Route15 0.254: v33.85,8.46 33.85,8.66
  other vias: 24.45,17.5 32.83,12.28 30.23,12.26 30.22,13.45 32.82,13.48 31.52,12.83 20.33,14.84 20.34,13.53 20.33,12.24 28.2,12.86 25.41,11.36 36.28,12.32 36.59,8.8 37.04,10.74 31.21,8.35 28.77,8.25 28.85,11.58 21.83,16.44
  pour Route2 (isolate 0.305, no thermals): -4.74,73 -4.74,-5 85.82,-5 85.82,73
  pour Top (no thermals): 19.46,10.69 19.46,16.29 21.66,18.49 25.06,18.49 26.86,16.69 37.66,16.69 37.66,7.69 26.06,7.69 23.66,10.09 20.06,10.09
  pour Route2 (isolate 0.305, no thermals): 94.99,37 94.99,69.5 84.49,69.5 84.49,37
IO0  (via drill 0.3)
  Top 0.152: Q3.3 50.21,13.65 54.41,9.45 U5.27 69.15,10.24 69.85,10.94 75.97,10.94 79.17,14.14 79.17,14.21 v79.11,14.27
  Route15 0.152: v79.11,14.27 83.58,18.74 83.58,36.56 88.47,40.68 89.8,40.68 J2.P$4
IO2
  Top 0.152: U5.38 83.12,2.61 N4.P4
IO4  (via drill 0.3)
  Top 0.152: U5.4 81.85,25.79 78.97,22.91 76.02,22.91 75.74,22.63 v75.74,12.9 v75.74,12.89
  Route15 0.152: v75.74,12.89 75.74,10.49 N3.P4
IO5  (via drill 0.3)
  Top 0.152: U5.5 80.58,25.34 78.45,23.21 75.89,23.21 75.07,22.39 75.07,12.27 v74.78,11.98
  Route15 0.152: v74.78,11.98 74.7,11.98 N3.P3
IO6  (via drill 0.3)
  Top 0.152: U5.6 79.31,25.35 77.78,23.82 76.07,23.82 74.28,22.03 74.28,12.57 v73.6,11.89
  Route15 0.152: v73.6,11.89 66.71,5 64.31,5 62.7,3.39 N3.P2
IO15  (via drill 0.3)
  Top 0.152: U5.8 76.77,24.99 73.42,21.64 73.42,12.87 v72.5,11.95
  Route15 0.152: v72.5,11.95 66.62,6.07 62.51,6.07 60.16,3.72 N3.P1
IO16  (via drill 0.3)
  Top 0.152: U5.9 75.5,24.42 72.69,21.61 72.69,13.57 v71.34,12.22
  Route15 0.152: v71.34,12.22 65.78,6.66 58.11,6.66 55.09,3.64 N5.P5
IO17  (via drill 0.3)
  Top 0.152: U5.10 74.23,24 72.24,22.01 72.24,14.6 69.91,12.27 v69.93,12.24
  Route15 0.152: v69.93,12.24 64.92,7.23 55.98,7.23 52.55,3.8 N5.P4
IO18  (via drill 0.3)
  Top 0.152: U5.11 73.32,26.59 73.32,23.59 71.74,22.01 71.74,15.56 v69.72,13.54 v69.7,13.55
  Route15 0.152: v69.7,13.55 64.06,7.91 54.28,7.91 50.01,3.64 N5.P3
IO19  (via drill 0.3)
  Top 0.152: U5.13 70.42,24.93 71.43,23.91 71.43,16.66 69.59,14.81 v69.48,14.91
  Route15 0.152: v69.48,14.91 63.03,8.46 52.26,8.46 47.47,3.67 N5.P2
IO20  (via drill 0.3)
  Top 0.152: U5.14 69.15,25.41 70.79,23.77 70.79,17.19 70.07,16.47 70.01,16.47 v69.97,16.51
  Route15 0.152: v69.97,16.51 64.24,10.78 64.24,10.74 62.62,9.12 50.09,9.12 44.93,3.96 N5.P1
IO38
  Top 0.152: U5.31 74.23,7.78 70.32,3.87 N3.P5
IO39
  Top 0.152: U5.32 75.5,7.09 72.87,4.46 N4.P0
IO40
  Top 0.152: U5.33 76.77,6.55 75.41,5.19 N4.P1
IO41
  Top 0.152: U5.34 78.04,2.61 N4.P2
IO42
  Top 0.152: U5.35 79.31,8.06 80.49,6.88 N4.P3
N$1
  Top 0.254: U10.4 11.17,9.11 | 11.17,9.11 11.13,9.15 10.99,9.29 | U10.6 11.3,8.11 11.14,8.27 11.14,9.08 11.17,9.11
  Top 0.813: D2.1 10.99,9.29 | 11.13,9.15 C61.1
N$2
  Top 0.305: R13.2 65.41,37.62 S1.1
N$3
  Top 0.152: R30.2 51.29,16.75 51.29,19.44 Q4.1
N$4
  Top 0.254: 29.97,17.8 R5.1 C15.2
  Top 0.305: U7.8 29.97,17.8 | R5.1 29.61,18.1 R3.2
N$5
  Top 0.508: 27.61,15.8 U7.10
  Top 0.61: 27.61,15.8 L1.1
  Top 0.813: L1.1 25.77,15.26 D1.1
N$6
  Top 0.305: U7.7 30.62,17.41 R5.2 32.16,18.95 C18.1
N$7
  Top 0.305: C15.1 31.53,20.41 R1.2
N$8
  Top 0.305: U1.4 39.08,41.55 C20.1
N$9
  Top 0.305: U1.5 38.02,40.91 C20.2
N$10
  Top 0.152: Q3.1 R29.2
N$11
  Top 0.254: R2.1 28.28,19.79 R3.1
N$17
  Top 0.152: R15.1 67.66,14.78 U5.23
N$24
  Top 0.254: Q8.1 46.32,9.7 R52.1
N$28
  Top 0.305: U1.17 50.54,36.35 C21.1
PD  (via drill 0.3)
  Top 0.152: v48.01,11.3 48.01,11.26 48.05,11.22 R52.2 49.5,9.67 R8.2 | v78.02,25.41 78.02,26.93 U5.7
  Bottom 0.152: v48.01,11.3 55.37,18.66 71.06,18.66 77.92,25.52 v78.02,25.41
PWR_DWN  (via drill 0.3)
  Top 0.152: R51.1 18.41,25.94 18.41,23.05 17.9,22.54 U3.3 17.15,21.43 v17.73,20.85 v17.72,20.84 | R50.1 34.98,18.2 | 34.98,18.2 34.16,17.38 33.44,17.38 33.23,17.16 U7.3 | 34.98,18.2 34.94,18.24 v34.94,20.43 36.81,20.43 38.14,19.1 38.14,13.85 41.34,10.65 Q8.3
  Route15 0.152: v17.72,20.84 34.55,20.84 34.94,20.46 v34.94,20.43
RGB  (via drill 0.35)
  Top 0.152: U5.39 84.41,9.47 84.41,10.44 82.82,12.02 82.04,12.02 v82.04,12.06 | v20.83,29.64 19.41,29.64 U11.4 18.47,29.81 16.95,31.33 16.95,32.22 17.74,33.01 U11.6
  Route15 0.152: v82.04,12.06 79.93,12.06 64.79,27.2 54.1,27.2 54.06,27.16 53.57,27.16 v52.61,28.12
  Bottom 0.152: v52.61,28.12 22.38,28.12 20.85,29.65 v20.83,29.64
RST_PD  (via drill 0.3, 0.4)
  Top 0.152: 48.55,38.32 U1.20 52.21,38.3 53.12,37.39 56.7,37.39 57.34,36.75 57.34,34.96 R14.1 59.73,32.57 v59.73,26.16 | v59.09,14.69 60.26,14.69 R15.2
  Route15 0.152: v59.73,26.16 59.73,15.41 59.05,14.73 v59.09,14.69
RTS
  Top 0.152: U6.14 47.77,19.71 R29.1 49.55,19.28 Q4.2
SCL  (via drill 0.3, 0.35)
  Top 0.152: U5.17 67.02,22.64 65.62,24.05 54.37,24.05 52.41,26.01 44.34,26.01 44.28,25.95 v44.28,25.93 | R34.1 40.61,24.95 38.37,22.71 38.02,22.71 v38.02,22.8 | v7.12,31.93 6.71,32.35 J3.4
  Top 0.203: R34.1 40.66,25.65 44,25.65 v44.28,25.93
  Route15 0.152: v44.28,25.93 41.01,22.66 41.01,10.11 36.21,5.31 32.44,5.31 29.68,2.55 N7.P1 | v38.02,22.8 35.38,25.44 35.38,27.23 32.02,30.59 8.47,30.59 v7.12,31.93
SCLK
  Top 0.152: U5.20 65.52,18.84 R7.1
SDA  (via drill 0.3, 0.35)
  Top 0.152: U5.12 71.69,27.83 71.16,28.36 66.96,28.36 63.05,24.45 54.71,24.45 52.27,26.89 43.48,26.89 v43.34,26.75 | v7.15,33.24 7.04,33.35 J3.3
  Top 0.203: R33.1 42.4,27.69 v43.34,26.75
  Route15 0.152: N7.P0 27.14,4.16 28.67,5.69 35.96,5.69 40.65,10.38 40.65,23.15 43.34,25.84 v43.34,26.75 36.45,26.75 32.14,31.06 9.33,31.06 v7.15,33.24
START
  Top 0.152: U5.24 67.88,13.73 R4.1
UCIPO
  Top 0.152: U1.13 41.31,35.7 R10.2
UCOPI  (via drill 0.3, 0.4)
  Top 0.152: R9.2 56.99,20.42 v56.01,19.44 55.09,18.52 55.09,15.02 v55.16,15.02 | v44.41,35.22 44.41,35.47 43.53,36.35 U1.12
  Route15 0.152: v56.01,19.44 55.93,19.44 44.41,30.95 v44.41,35.22 | v55.16,15.02 55.16,14.06 51.67,10.57 42.81,10.57 N7.P3
UCS  (via drill 0.4)
  Top 0.152: R6.2 55.12,22.41 52.59,24.94 46.35,24.94 v46.23,25.06 45.25,25.06 R12.1 | 42.67,37.64 42.65,37.66 41.83,37.66 40.66,36.49 v39.74,36.49
  Top 0.2: 42.64,37.6 42.67,37.64 U1.10
  Route15 0.152: v46.23,25.06 40.54,30.75 38.42,30.75 37.29,31.88 37.29,34.01 39.74,36.46 v39.74,36.49
UDRDY
  Top 0.152: R11.2 42.09,34.87 42.51,34.87 U1.14
USCLK  (via drill 0.3, 0.4)
  Top 0.152: U1.11 42.66,36.97 44.24,36.97 v44.31,36.9 | R7.2 58.33,18.42 57.51,19.24 v57.51,19.32 57.51,19.07 55.99,17.55 55.99,15.26 v56.31,14.94
  Route15 0.152: v57.51,19.32 57.51,19.84 47.23,30.12 47.23,33.38 45.87,34.74 45.87,35.34 v44.31,36.9 | v56.31,14.94 56.31,14.31 51.91,9.91 43.9,9.91 37.3,3.31 N7.P4
USTART  (via drill 0.3, 0.35)
  Top 0.152: R4.2 63.71,13.73 62.96,12.98 v58.5,12.98 58.5,12.78 R16.2
  Top 0.2: U1.9 43.72,38.3 44.02,38 v44.21,38
  Route15 0.152: v58.5,12.98 58.45,13.03 58.45,19.77 47.55,30.67 47.55,33.65 46.62,34.58 46.62,35.59 v44.21,38
V+  (via drill 0.4)
  Top 0.254: U1.6 44.27,40.26 45.58,38.94 45.58,34.02 C44.1
  Top 0.305: 46.18,31.18 C23.1 46.24,31.24 | 46.18,31.18 46.14,31.14 | v24.25,29.7 21.52,26.97 C4.1 | v45.09,31.18 46.18,31.18
  Top 0.406: 46.34,31.26 C23.1 46.31,31.21 | 46.34,33.29 C44.1
  Top 0.508: 46.34,31.26 46.34,33.29
  Top 0.61: U3.5 20.8,24.44 20.95,24.29 21.41,24.29 C4.1
  Bottom 0.305: v24.25,29.7 24.25,30 25.22,30.98 44.9,30.98 v45.09,31.18
V-  (via drill 0.3, 0.35)
  Top 0.152: C25.1 38.19,39.78
  Top 0.254: C25.1 38.13,40.15 | U1.7 44.32,39.6 45.17,38.75 45.17,33.85 C44.2
  Top 0.305: 37.26,39.78 v37.19,39.71 v37.2,39.7 | v32.18,25.14 34.47,25.14 42.62,33.29 C44.2
  Top 0.406: U1.7 40.66,39.6 C22.2 C25.1 | U4.3 31.07,25.09 C1.1 | 38.19,39.78 37.26,39.78
  Top 0.508: C1.1 31.15,24.8 31.84,24.8 v32.18,25.14
  Bottom 0.305: 18.03,39.7 U$10.P$1 6.54,43.27 U$11.N1
  Bottom 0.406: v37.2,39.7 18.03,39.7
  Bottom 0.508: v32.18,25.14 32.1,25.06
VBUS  (via drill 0.3)
  Top 0.254: J1.B9 5.53,19.45 v5.35,19.63 v5.35,19.64 | v8.95,19.64 8.89,19.7 J1.A4 | J1.A9 8.14,16.7 | 8.14,16.7 9.46,16.7 | J1.B4 7.13,16.95 7.4,16.68 8.12,16.68 8.14,16.7
  Top 0.305: C47.1 10.23,17.47 9.46,16.7
  Top 0.406: v8.95,19.64 10.73,19.64 C57.1
  Top 0.813: C47.1 10.81,17.54 C57.1 10.84,19.75 C56.1 12.86,19.71 FB1.1
  Route15 0.254: v5.35,19.64 v5.36,19.65 v8.94,19.65 v8.95,19.64
  Bottom 0.61: v8.95,19.64 10.03,19.64 10.67,19 10.67,3.76 N6.P0
VCC_LP
  Top 0.152: 17.52,24.44 U3.1 17.06,24.53 R51.2 17.06,27.14 17.88,27.96 20.73,27.96 23.43,30.66 32.97,30.66 34.63,29 34.63,26.96 34.14,26.47 U4.4
  Top 0.305: U3.1 17.1,24.4 | L3.1 12.51,26.03 C49.1 12.57,24.47 C3.1
  Top 0.508: C3.1 17.1,24.4
  Top 0.813: C3.1 15.26,24.44
VREF_2.5  (via drill 0.35)
  Top 0.203: 44.02,38.95 v44.03,38.94
  Top 0.406: 44.02,38.95 U1.8 42.68,38.97 41.69,38.97 40.8,38.08 C22.1
  Bottom 0.254: v44.03,38.94 43.89,38.8
  Bottom 0.305: 16.48,38.8 4.61,38.8 U$11.N2
  Bottom 0.406: 43.89,38.8 16.48,38.8
VREF_2.048  (via drill 0.35)
  Top 0.203: v68.93,37.03 67.94,37.03 R13.1
  Top 0.305: C8.1 67.92,37.02 R13.1
  Top 0.406: 72.46,38.77 U2.6 69.98,38.77 C46.1 C8.1 67.86,38.78
  Bottom 0.203: N1.P0 75.93,44.03 v68.93,37.03
VSS  (via drill 0.4)
  Top 0.152: U7.9 29.32,14.44 28.71,13.82 26.51,13.82 25.31,12.62 D1.2
  Top 0.203: R2.2 25.94,20.21 23.76,18.03 23.22,18.03 v23.12,17.93
  Top 0.305: 27.49,21.12 R2.2 28.78,22.41 R1.1
  Top 0.406: v23.12,17.93 23.37,17.68 | C12.1 23.37,14.71
  Top 0.508: v23.12,17.93 23.12,21.32 25.3,23.5 L4.2
  Top 0.813: 24.91,12.62 D1.2 C13.1 | 23.37,17.68 23.37,14.71 | 25.12,25.57 L4.2
  Top 1.016: C13.1 23.22,14.56 C12.1
VSS_LP
  Top 0.406: C2.1 29.67,27.12 U4.2
  Top 0.508: L4.1 26.92,27.45 C42.1 29.13,27.02 C2.1

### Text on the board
tNames: GND | AINCOM | AIN9 | AIN8 | AIN7 | AIN6 | AIN5 | AIN4 | AIN3 | AIN2 | AIN1 | AIN0 | GND | AIN4 / Direct | AIN8 / Direct | AIN6 / Direct | AIN2 / Direct | AINCOM | GND | GND | -2.5V | -2.5V | 2 | 2.048V | 2.5V Ref | . | 1 | IoT Precision Logger / by Anabit V1.1 | I2C & 3V3 | Dip Switch / 1 A0 = 2.048V Ref / 2 A1 = AGND | IO2 | 3V3 | GND | GND | RST | SDA | SCL | GND | COPI | CIPO | GND | IO20 | IO19 | IO18 | IO17 | IO16 | GND | IO15 | IO6 | IO5 | IO4 | IO38 | IO39 | IO40 | IO41 | IO42 | GND | GND | SCLK | VIN
bNames: GND | AINCOM | AIN9 | AIN8 | AIN7 | AIN6 | AIN5 | AIN4 | AIN3 | AIN2 | AIN1 | AIN0 | IoT Precision Logger / ESP32+ADC+PGA+MUX / by Anabit V1.1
